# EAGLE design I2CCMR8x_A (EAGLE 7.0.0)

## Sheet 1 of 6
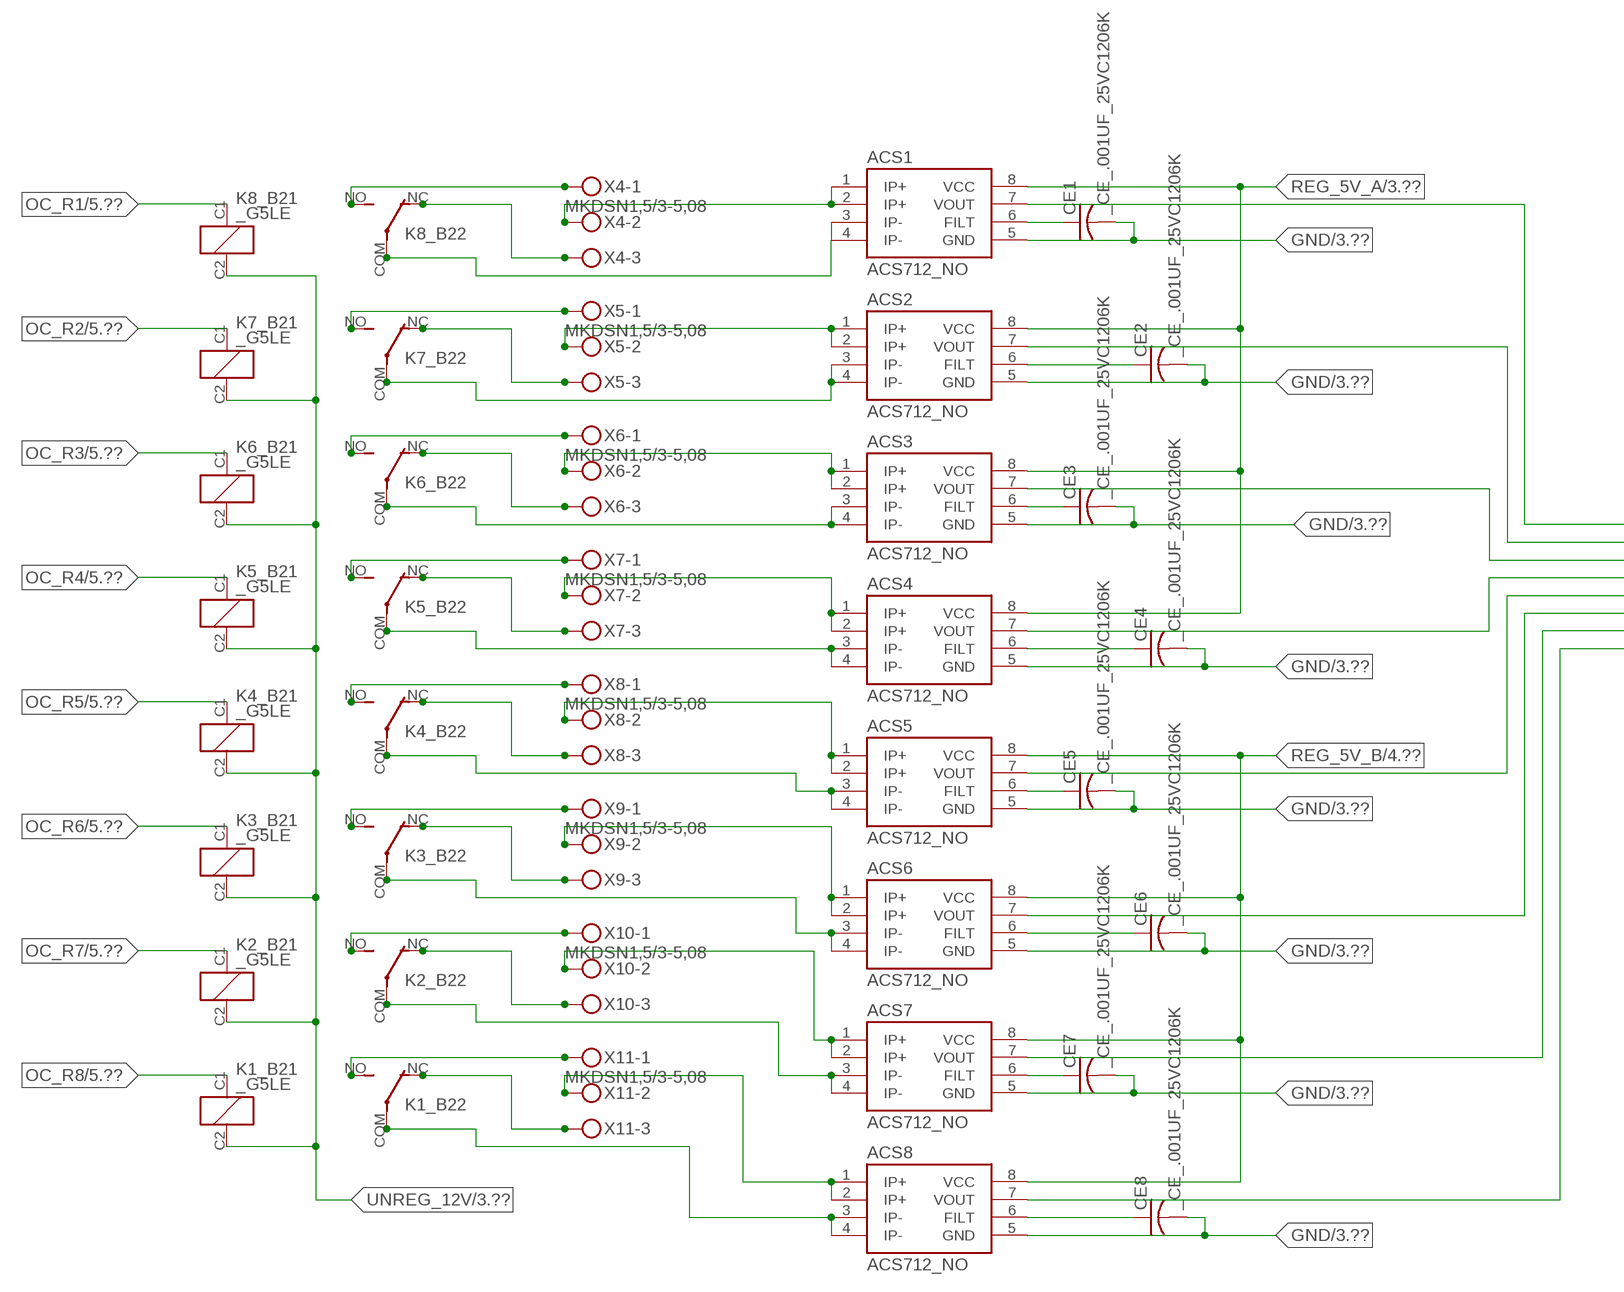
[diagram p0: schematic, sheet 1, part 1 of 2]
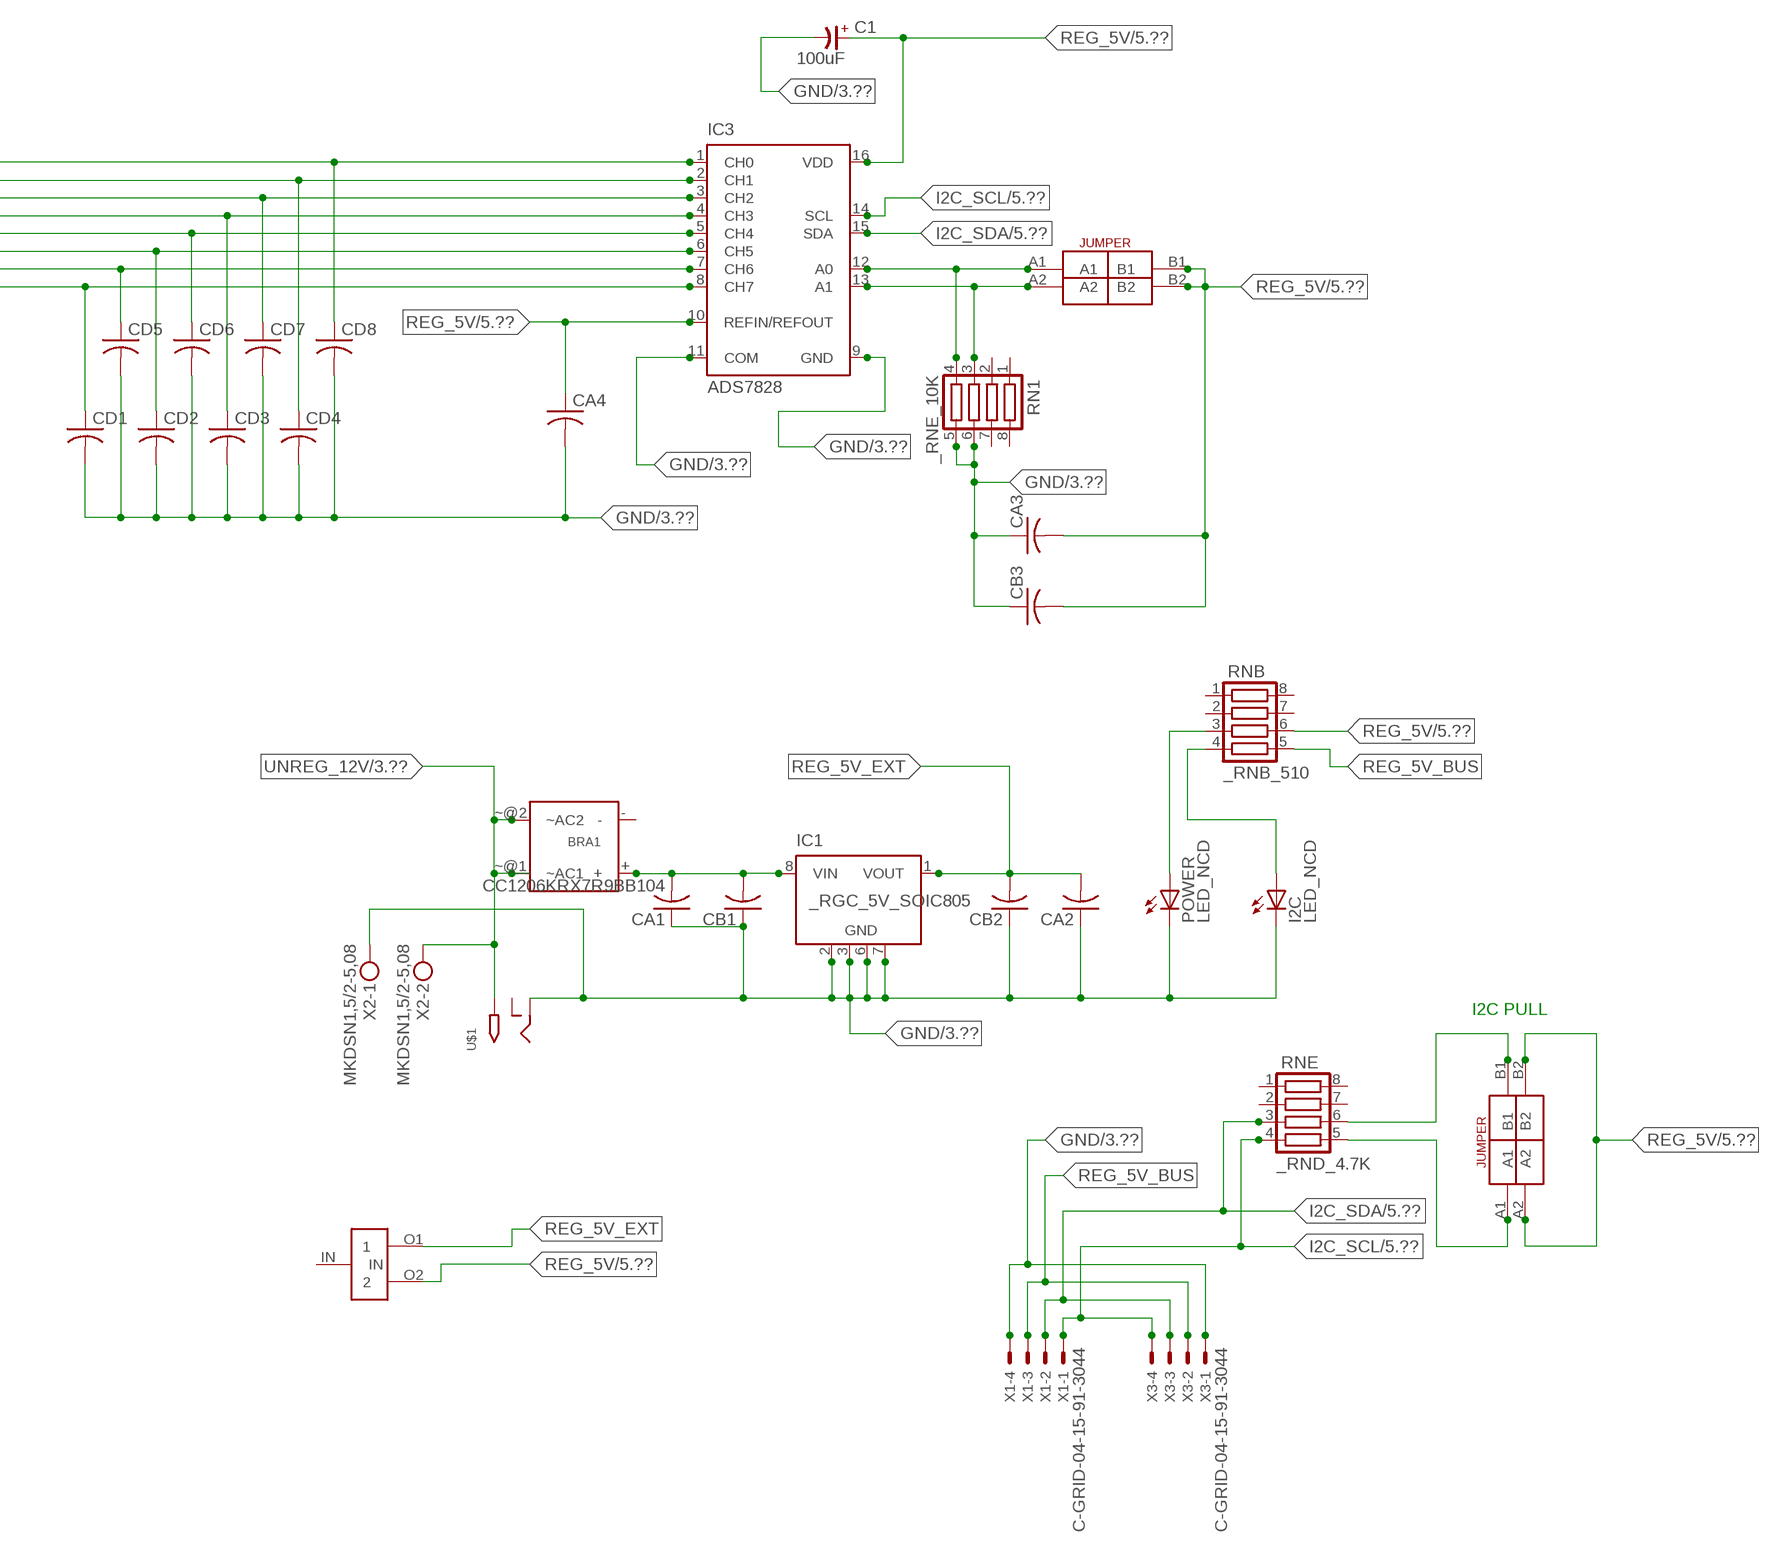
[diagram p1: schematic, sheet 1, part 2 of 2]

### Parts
ACS1  ACS712_NO  [_MA_DUAL_N-FET]
ACS2  ACS712_NO  [_MA_DUAL_N-FET]
ACS3  ACS712_NO  [_MA_DUAL_N-FET]
ACS4  ACS712_NO  [_MA_DUAL_N-FET]
ACS5  ACS712_NO  [_MA_DUAL_N-FET]
ACS6  ACS712_NO  [_MA_DUAL_N-FET]
ACS7  ACS712_NO  [_MA_DUAL_N-FET]
ACS8  ACS712_NO  [_MA_DUAL_N-FET]
BRA1  MB2S_  [MB2S]
C1  100uF  CP-E-025X060  [E-025X060]
CA1  CC1206KRX7R9BB104  [.1UF]
CA2  CC1206KRX7R9BB104C1206K  [CC1206KRX7R9BB104]
CA3  CC1206KRX7R9BB104C1206K  [CC1206KRX7R9BB104]
CA4  CC1206KRX7R9BB104C1206K  [CC1206KRX7R9BB104]
CB1  TMK316F106ZL-TC1206K  [TMK316F106ZL-T]
CB2  TMK316F106ZL-TC1206K  [TMK316F106ZL-T]
CB3  TMK316F106ZL-TC1206K  [TMK316F106ZL-T]
CD1  _CD_10NF_50VC1206K  [_CD_10NF_50V]
CD2  _CD_10NF_50VC1206K  [_CD_10NF_50V]
CD3  _CD_10NF_50VC1206K  [_CD_10NF_50V]
CD4  _CD_10NF_50VC1206K  [_CD_10NF_50V]
CD5  _CD_10NF_50VC1206K  [_CD_10NF_50V]
CD6  _CD_10NF_50VC1206K  [_CD_10NF_50V]
CD7  _CD_10NF_50VC1206K  [_CD_10NF_50V]
CD8  _CD_10NF_50VC1206K  [_CD_10NF_50V]
CE1  _CE_.001UF_25VC1206K  [CE]
CE2  _CE_.001UF_25VC1206K  [CE]
CE3  _CE_.001UF_25VC1206K  [CE]
CE4  _CE_.001UF_25VC1206K  [CE]
CE5  _CE_.001UF_25VC1206K  [CE]
CE6  _CE_.001UF_25VC1206K  [CE]
CE7  _CE_.001UF_25VC1206K  [CE]
CE8  _CE_.001UF_25VC1206K  [CE]
I2C  LED_NCD  [CHIPLED_0603]
IC1  _RGC_5V_SOIC805  [_RGC_5V_SOIC8]
IC3  ADS7828  [TSSOP16-PW]
K1_B2  _G5LE  [G5LE]
K2_B2  _G5LE  [G5LE]
K3_B2  _G5LE  [G5LE]
K4_B2  _G5LE  [G5LE]
K5_B2  _G5LE  [G5LE]
K6_B2  _G5LE  [G5LE]
K7_B2  _G5LE  [G5LE]
K8_B2  _G5LE  [G5LE]
POWER  LED_NCD  [CHIPLED_0603]
RN1  _RNE_10K  [RNE]
RNB  _RNB_510  [RNB]
RNE  _RND_4.7K  [RND]
U$1  2.1MMJACK  [PJ-102A]
U$2  LINK_2  [LINK_2]
U$3  JUMPER_2X2  [JUMPER_2X2]
U$4  JUMPER_2X2  [JUMPER_2X2]
X1  C-GRID-04-15-91-3044  [15-91-04]
X2  MKDSN1,5/2-5,08  [MKDSN1,5/2-5,08]
X3  C-GRID-04-15-91-3044  [15-91-04]
X4  MKDSN1,5/3-5,08  [MKDSN1,5/3-5,08]
X5  MKDSN1,5/3-5,08  [MKDSN1,5/3-5,08]
X6  MKDSN1,5/3-5,08  [MKDSN1,5/3-5,08]
X7  MKDSN1,5/3-5,08  [MKDSN1,5/3-5,08]
X8  MKDSN1,5/3-5,08  [MKDSN1,5/3-5,08]
X9  MKDSN1,5/3-5,08  [MKDSN1,5/3-5,08]
X10  MKDSN1,5/3-5,08  [MKDSN1,5/3-5,08]
X11  MKDSN1,5/3-5,08  [MKDSN1,5/3-5,08]

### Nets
GND: ACS1.5(GND) ACS2.5(GND) ACS3.5(GND) ACS4.5(GND) ACS5.5(GND) ACS6.5(GND) ACS7.5(GND) ACS8.5(GND) C1.- CA1.1 CA2.1 CA3.1 CA4.2 CB1.1 CB2.1 CB3.1 CD1.2 CD2.2 CD3.2 CD4.2 CD5.2 CD6.2 CD7.2 CD8.2 CE1.2 CE2.2 CE3.2 CE4.2 CE5.2 CE6.2 CE7.2 CE8.2 I2C.C IC1.2(GND) IC1.3(GND) IC1.6(GND) IC1.7(GND) IC3.9(GND) IC3.11(COM) POWER.C RN1.5 RN1.6 U$1.RING X1.4 X2.1 X3.1 ; also sheet 3,4,5
I2C_SCL: IC3.14(SCL) RNE.4 X1.1 X3.4 ; also sheet 5
I2C_SDA: IC3.15(SDA) RNE.3 X1.2 X3.3 ; also sheet 5
N$1: BRA1.+ CA1.2 CB1.2 IC1.8(VIN)
N$2: POWER.A RNB.3
N$3: I2C.A RNB.4
N$4: RNE.5 U$3.A1
N$5: RNE.6 U$3.B1
N$6: ACS5.7(VOUT) CD6.1 IC3.5(CH4)
N$7: ACS1.1(IP+) ACS1.2(IP+) X4.2
N$9: ACS1.7(VOUT) CD8.1 IC3.1(CH0)
N$10: ACS2.7(VOUT) CD4.1 IC3.2(CH1)
N$11: ACS3.7(VOUT) CD7.1 IC3.3(CH2)
N$12: ACS4.7(VOUT) CD3.1 IC3.4(CH3)
N$13: ACS2.1(IP+) ACS2.2(IP+) X5.2
N$14: ACS6.7(VOUT) CD2.1 IC3.6(CH5)
N$15: ACS7.7(VOUT) CD5.1 IC3.7(CH6)
N$17: IC3.12(A0) RN1.4 U$4.A1
N$18: IC3.13(A1) RN1.3 U$4.A2
N$21: ACS4.1(IP+) ACS4.2(IP+) X7.2
N$22: ACS4.3(IP-) ACS4.4(IP-) K5_B2.COM(2:COM)
N$23: ACS5.1(IP+) ACS5.2(IP+) X8.2
N$24: ACS7.1(IP+) ACS7.2(IP+) X10.2
N$25: ACS6.1(IP+) ACS6.2(IP+) X9.2
N$29: ACS8.1(IP+) ACS8.2(IP+) X11.2
N$33: ACS1.6(FILT) CE1.1
N$34: ACS2.6(FILT) CE2.1
N$35: ACS3.6(FILT) CE3.1
N$36: ACS4.6(FILT) CE4.1
N$37: ACS8.7(VOUT) CD1.1 IC3.8(CH7)
N$38: ACS5.6(FILT) CE5.1
N$39: ACS6.6(FILT) CE6.1
N$40: ACS7.6(FILT) CE7.1
N$41: ACS8.6(FILT) CE8.1
N$42: ACS1.3(IP-) ACS1.4(IP-) K8_B2.COM(2:COM)
N$43: K8_B2.NC(2:NC) X4.3
N$44: K8_B2.NO(2:NO) X4.1
N$45: K7_B2.NO(2:NO) X5.1
N$46: K6_B2.NO(2:NO) X6.1
N$137: K7_B2.NC(2:NC) X5.3
N$138: ACS2.3(IP-) ACS2.4(IP-) K7_B2.COM(2:COM)
N$139: K6_B2.NC(2:NC) X6.3
N$140: ACS3.3(IP-) ACS3.4(IP-) K6_B2.COM(2:COM)
N$141: K5_B2.NC(2:NC) X7.3
N$143: K5_B2.NO(2:NO) X7.1
N$144: K4_B2.NO(2:NO) X8.1
N$145: K4_B2.NC(2:NC) X8.3
N$146: ACS5.3(IP-) ACS5.4(IP-) K4_B2.COM(2:COM)
N$147: K3_B2.NO(2:NO) X9.1
N$148: K3_B2.NC(2:NC) X9.3
N$149: ACS6.3(IP-) ACS6.4(IP-) K3_B2.COM(2:COM)
N$150: K2_B2.NO(2:NO) X10.1
N$151: K2_B2.NC(2:NC) X10.3
N$152: ACS7.3(IP-) ACS7.4(IP-) K2_B2.COM(2:COM)
N$153: K1_B2.NO(2:NO) X11.1
N$154: K1_B2.NC(2:NC) X11.3
N$155: ACS8.3(IP-) ACS8.4(IP-) K1_B2.COM(2:COM)
N$166: ACS3.1(IP+) ACS3.2(IP+) X6.2
OC_R1: K8_B2.C1(1:C1) ; also sheet 5
OC_R2: K7_B2.C1(1:C1) ; also sheet 5
OC_R3: K6_B2.C1(1:C1) ; also sheet 5
OC_R4: K5_B2.C1(1:C1) ; also sheet 5
OC_R5: K4_B2.C1(1:C1) ; also sheet 5
OC_R6: K3_B2.C1(1:C1) ; also sheet 5
OC_R7: K2_B2.C1(1:C1) ; also sheet 5
OC_R8: K1_B2.C1(1:C1) ; also sheet 5
REG_5V: C1.+ CA3.2 CA4.1 CB3.2 IC3.10(REFIN/REFOUT) IC3.16(VDD) RNB.6 U$2.O2 U$3.A2 U$3.B2 U$4.B1 U$4.B2 ; also sheet 5
REG_5V_A: ACS1.8(VCC) ACS2.8(VCC) ACS3.8(VCC) ACS4.8(VCC) ; also sheet 3
REG_5V_B: ACS5.8(VCC) ACS6.8(VCC) ACS7.8(VCC) ACS8.8(VCC) ; also sheet 4
REG_5V_BUS: RNB.5 X1.3 X3.2
REG_5V_EXT: CA2.2 CB2.2 IC1.1(VOUT) U$2.O1
UNREG_12V: BRA1.~@1(~AC1) BRA1.~@2(~AC2) K1_B2.C2(1:C2) K2_B2.C2(1:C2) K3_B2.C2(1:C2) K4_B2.C2(1:C2) K5_B2.C2(1:C2) K6_B2.C2(1:C2) K7_B2.C2(1:C2) K8_B2.C2(1:C2) U$1.TIP X2.2 ; also sheet 3,4,5
Unconnected: BRA1.- IC1.4(NC) IC1.5(NC) RN1.1 RN1.2 RN1.7 RN1.8 RNB.1 RNB.2 RNB.7 RNB.8 RNE.1 RNE.2 RNE.7 RNE.8 U$1.RING_SW U$2.IN

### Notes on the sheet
- I2C PULL

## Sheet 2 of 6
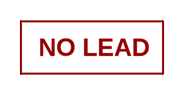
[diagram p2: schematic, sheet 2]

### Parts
U$16  NOPB_LOGO_SYM  [NOPB_LOGO_SYM]

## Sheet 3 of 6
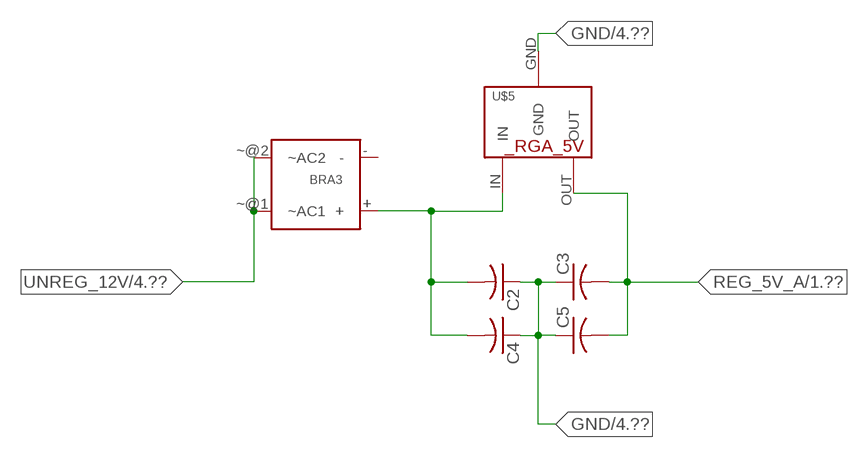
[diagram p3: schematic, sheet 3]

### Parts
BRA3  MB2S_  [MB2S]
C2  _CA_.10UF_50VC1206K  [_CA_.1UF_50V]
C3  _CA_.10UF_50VC1206K  [_CA_.1UF_50V]
C4  _CB_10UF_25VC1206K  [_CB_10UF_25V]
C5  _CB_10UF_25VC1206K  [_CB_10UF_25V]
U$5  _RGA_5V  [_RGA_5V]

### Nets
GND: C2.1 C3.1 C4.1 C5.1 U$5.GND ; also sheet 1,4,5
N$31: BRA3.+ C2.2 C4.2 U$5.IN
REG_5V_A: C3.2 C5.2 U$5.OUT ; also sheet 1
UNREG_12V: BRA3.~@1(~AC1) BRA3.~@2(~AC2) ; also sheet 1,4,5
Unconnected: BRA3.-

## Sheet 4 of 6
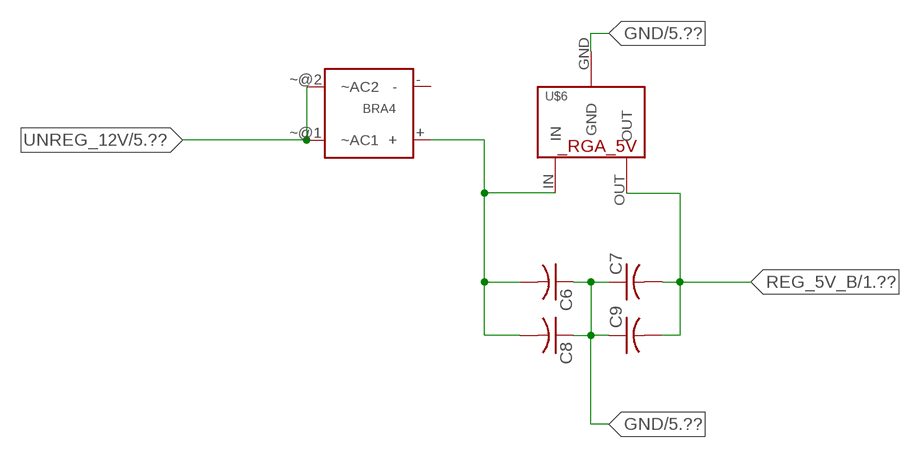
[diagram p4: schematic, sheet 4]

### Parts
BRA4  MB2S_  [MB2S]
C6  _CA_.10UF_50VC1206K  [_CA_.1UF_50V]
C7  _CA_.10UF_50VC1206K  [_CA_.1UF_50V]
C8  _CB_10UF_25VC1206K  [_CB_10UF_25V]
C9  _CB_10UF_25VC1206K  [_CB_10UF_25V]
U$6  _RGA_5V  [_RGA_5V]

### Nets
GND: C6.1 C7.1 C8.1 C9.1 U$6.GND ; also sheet 1,3,5
N$32: BRA4.+ C6.2 C8.2 U$6.IN
REG_5V_B: C7.2 C9.2 U$6.OUT ; also sheet 1
UNREG_12V: BRA4.~@1(~AC1) BRA4.~@2(~AC2) ; also sheet 1,3,5
Unconnected: BRA4.-

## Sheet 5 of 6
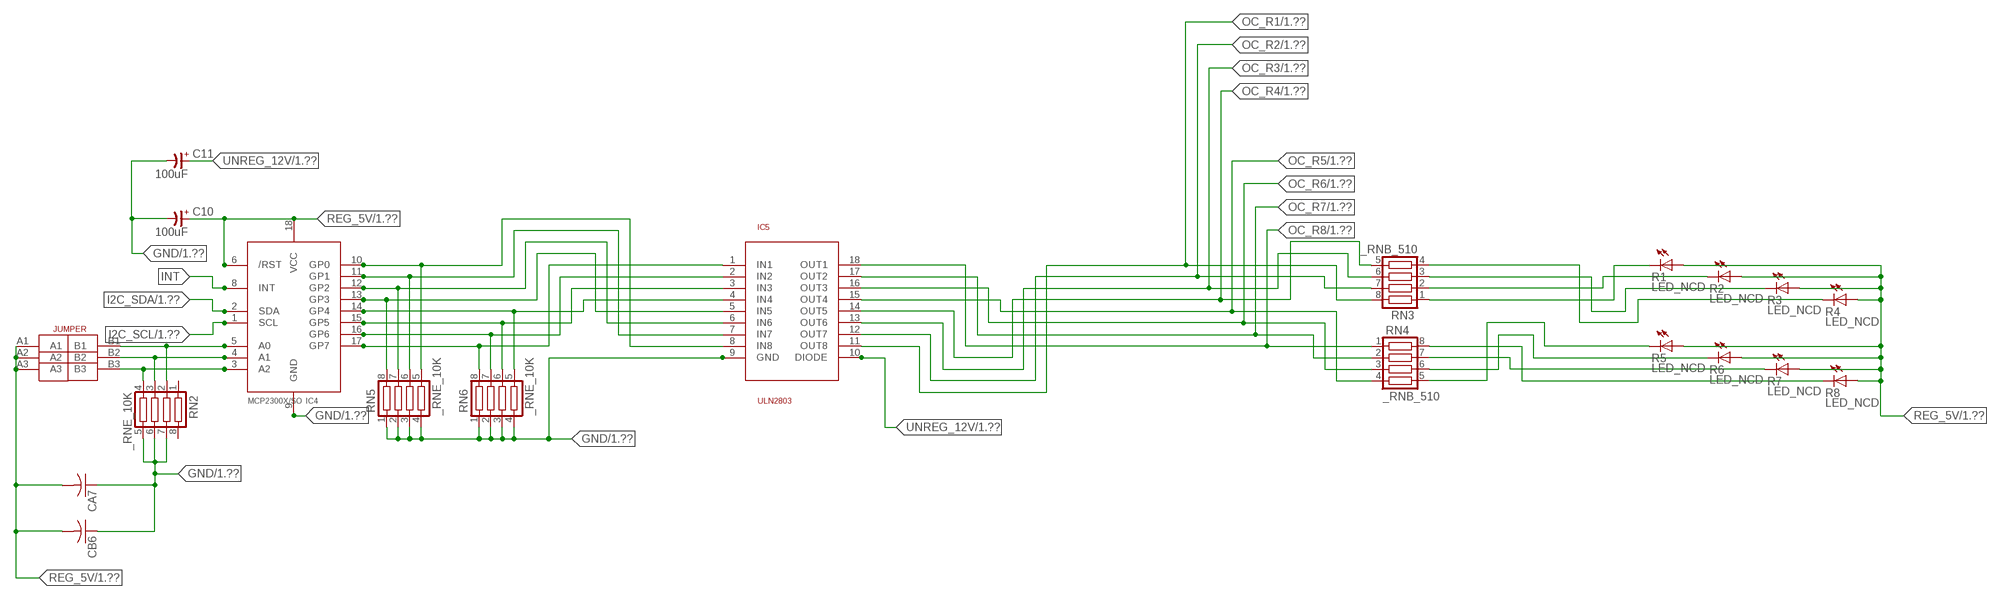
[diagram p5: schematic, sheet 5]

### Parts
C10  100uF  CP-E-025X060  [E-025X060]
C11  100uF  CP-E-025X060  [E-025X060]
CA7  CC1206KRX7R9BB104C1206K  [CC1206KRX7R9BB104]
CB6  TMK316F106ZL-TC1206K  [TMK316F106ZL-T]
IC4  MCP2300X/SO  [SO18W]
IC5  ULN2803  [SO18L]
R1  LED_NCD  [CHIPLED_0603]
R2  LED_NCD  [CHIPLED_0603]
R3  LED_NCD  [CHIPLED_0603]
R4  LED_NCD  [CHIPLED_0603]
R5  LED_NCD  [CHIPLED_0603]
R6  LED_NCD  [CHIPLED_0603]
R7  LED_NCD  [CHIPLED_0603]
R8  LED_NCD  [CHIPLED_0603]
RN2  _RNE_10K  [RNE]
RN3  _RNB_510  [RNB]
RN4  _RNB_510  [RNB]
RN5  _RNE_10K  [RNE]
RN6  _RNE_10K  [RNE]
U$18  JUMPER_3X2  [JUMPER_3X2]

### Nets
GND: C10.- C11.- CA7.1 CB6.1 IC4.9(GND) IC5.9(GND) RN2.5 RN2.6 RN2.7 RN5.1 RN5.2 RN5.3 RN5.4 RN6.1 RN6.2 RN6.3 RN6.4 ; also sheet 1,3,4
GP4: IC4.14(GP4) IC5.4(IN4) RN6.5
GP6: IC4.16(GP6) IC5.2(IN2) RN6.7
I2C_SCL: IC4.1(SCL) ; also sheet 1
I2C_SDA: IC4.2(SDA) ; also sheet 1
INT: IC4.8(INT)
N$47: IC4.5(A0) RN2.2 U$18.B1
N$48: IC4.4(A1) RN2.3 U$18.B2
N$49: IC4.3(A2) RN2.4 U$18.B3
N$50: IC4.12(GP2) IC5.6(IN6) RN5.7
N$51: IC4.11(GP1) IC5.7(IN7) RN5.6
N$52: IC4.10(GP0) IC5.8(IN8) RN5.5
N$53: R1.C RN3.1
N$54: R2.C RN3.2
N$55: R3.C RN3.3
N$56: R4.C RN3.4
N$57: R8.C RN4.8
N$81: R7.C RN4.7
N$82: R6.C RN4.6
N$83: R5.C RN4.5
N$89: IC4.13(GP3) IC5.5(IN5) RN5.8
N$93: IC4.15(GP5) IC5.3(IN3) RN6.6
N$94: IC4.17(GP7) IC5.1(IN1) RN6.8
OC_R1: IC5.11(OUT8) RN3.8 ; also sheet 1
OC_R2: IC5.12(OUT7) RN3.7 ; also sheet 1
OC_R3: IC5.13(OUT6) RN3.6 ; also sheet 1
OC_R4: IC5.14(OUT5) RN3.5 ; also sheet 1
OC_R5: IC5.15(OUT4) RN4.4 ; also sheet 1
OC_R6: IC5.16(OUT3) RN4.3 ; also sheet 1
OC_R7: IC5.17(OUT2) RN4.2 ; also sheet 1
OC_R8: IC5.18(OUT1) RN4.1 ; also sheet 1
REG_5V: C10.+ CA7.2 CB6.2 IC4.6(/RST) IC4.18(VCC) R1.A R2.A R3.A R4.A R5.A R6.A R7.A R8.A U$18.A1 U$18.A2 U$18.A3 ; also sheet 1
UNREG_12V: C11.+ IC5.10(DIODE) ; also sheet 1,3,4
Unconnected: RN2.1 RN2.8

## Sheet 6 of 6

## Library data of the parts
ACS1-ACS8 = NCD_ULTIMATE_LIBRARY:ACS712_NO: Semiconductor Sensor Current Hall-effect-based isolated linear current sensor Digikey 620-1190-2-ND/ACS712ELCTR-20A-T
BRA1 BRA3 BRA4 = NCD_ULTIMATE_LIBRARY:MB2S: Bridge Rectifier BRA MB2S 200V 500ma Digikey MB2S-TPMSTR-ND/MB2S-TP
C1 C10 C11 = NCD_ULTIMATE_LIBRARY:CP-: Capacitors All Kinds POLARIZED CAP
C2 C3 C6 C7 = NCD_ULTIMATE_LIBRARY:_CA_.10UF_50V: Capacitor .1uF SMT
C4 C5 C8 C9 = NCD_ULTIMATE_LIBRARY:_CB_10UF_25V: Capacitor 10uF SMT
CA1-CA4 CA7 = NCD_ULTIMATE_LIBRARY:CC1206KRX7R9BB104: Capacitor CA .1uF 50V SMT C1206K CC1206KRX7R9BB104
CB1-CB3 CB6 = NCD_ULTIMATE_LIBRARY:TMK316F106ZL-T: Capacitor CB 10uF SMT 1206 TMK316F106ZL-T
CD1-CD8 = NCD_ULTIMATE_LIBRARY:_CD_10NF_50V: Capacitor 10nF SMT
CE1-CE8 = NCD_ULTIMATE_LIBRARY:_CE_.001UF_25V: Capacitor .001uF SMT
I2C POWER = NCD_ULTIMATE_bhaskar:LED_NCD
IC1 = NCD_ULTIMATE_LIBRARY:_RGC_5V_SOIC8: Regulator Linear 5V Chip Positive VOLTAGE REGULATOR Digikey 497-7267-2-ND/L78L05CD13TR
IC3 = NCD_ULTIMATE_LIBRARY:ADS7828: Semiconductor ADC I2C 12-Bit, 8-Channel Sampling ANALOG-TO-DIGITAL CONVERTER Digikey 296-12402-2-ND Source: www.ti.com .. ADS7828.pdf / ADS7828E/250; MF: TEXAS INSTRUMENTS; MPN: ADS7828E/250; OC_FARNELL: 1470338; OC_NEWARK: 74C7158
IC4 = NCD_ULTIMATE_LIBRARY:MCP2300X: Semiconductor Port Expander I/O 8-Bit I2C MCP23008 Inexpensive i2c i/o expander - 8 general purpose i/o pins with optional pullups
IC5 = NCD_ULTIMATE_LIBRARY:ULN2803: Semiconductor 8 O.C. N-Channel Transistor Driver Digikey ULN2803AFWGCELTR-ND/ULN2803AFWG,C,EL
K1_B2 K2_B2 K3_B2 K4_B2 K5_B2 K6_B2 K7_B2 K8_B2 = NCD_ULTIMATE_LIBRARY:_G5LE: Relay 5A/10A SPDT; OC_FARNELL: unknown; OC_NEWARK: unknown
R1-R8 = NCD_ULTIMATE_LIBRARY:LED_NCD: LED Digikey 754-1132-2-ND/APT2012SRCPRV
RN1 RN2 RN5 RN6 = NCD_ULTIMATE_LIBRARY:_RNE_10K: Resistor Array RNE SMT 10K x 4 Single Resistor Source: http://www.ctscorp.com/components/Datasheets/CTSChipArrayDs.pdf Digikey 742C083103JPTR-ND/742C083103JP; OC_FARNELL: unknown; OC_NEWARK: unknown
RN3 RN4 RNB = NCD_ULTIMATE_LIBRARY:_RNB_510: Resistor Array RNB SMT 510 x 4 Single Resistor Source: http://www.ctscorp.com/components/Datasheets/CTSChipArrayDs.pdf Digikey 742C083511JPTR-ND/ 742C083511JP; OC_FARNELL: unknown; OC_NEWARK: unknown
RNE = NCD_ULTIMATE_LIBRARY:_RND_4.7K: Resistor Array RND SMT 4.7K x 4 Single Resistor Source: http://www.ctscorp.com/components/Datasheets/CTSChipArrayDs.pdf Digikey 742C083472JPTR-ND/742C083472JP; OC_FARNELL: unknown; OC_NEWARK: unknown
U$1 = NCD_ULTIMATE_CONNECTORS:2.1MMJACK: 2.1mm x 5.5mm DC jack with internal switch. Digikey part #PJ-102A, 4UCON part #05537 By microbuilder.eu
U$2 = NCD_ULTIMATE_LIBRARY:LINK_2: PAD_top
U$3 U$4 = NCD_ULTIMATE_CONNECTORS:JUMPER_2X2
U$5 U$6 = NCD_ULTIMATE_LIBRARY:_RGA_5V: Regulator Linear 5V Digikey 497-7255-2-ND/ L7805CDT-TR
U$16 = PatternAgents-Logos:NOPB_LOGO_SYM: NOPB_LOGO_SYM
U$18 = NCD_ULTIMATE_CONNECTORS:JUMPER_3X2
X1 X3 = NCD_ULTIMATE_CONNECTORS:C-GRID-04: CONNECTOR 4-Pos I2C wire to board 2.54 mm (0.100") pitch header Digikey WM1342-ND/0015912045; OC_FARNELL: unknown; OC_NEWARK: unknown
X2 = NCD_ULTIMATE_CONNECTORS:MKDSN1,5/2-5,08: MKDSN 1,5/ 2-5,08 Printklemme
X4-X11 = NCD_ULTIMATE_CONNECTORS:MKDSN1,5/3-5,08: MKDSN 1,5/ 3-5,08 Printklemme Nennstrom: 13,5 A Nennspannung: 250 V Rastermaß: 5,08 mm Polzahl: 3 Anschlussart: Schraubanschluss Montage: Löten Anschlussrichtung Leiter/Platine: 0 ° Artikelnummer: 1729131 Source: http://eshop.phoenixcontact.com .. 1729131.pdf

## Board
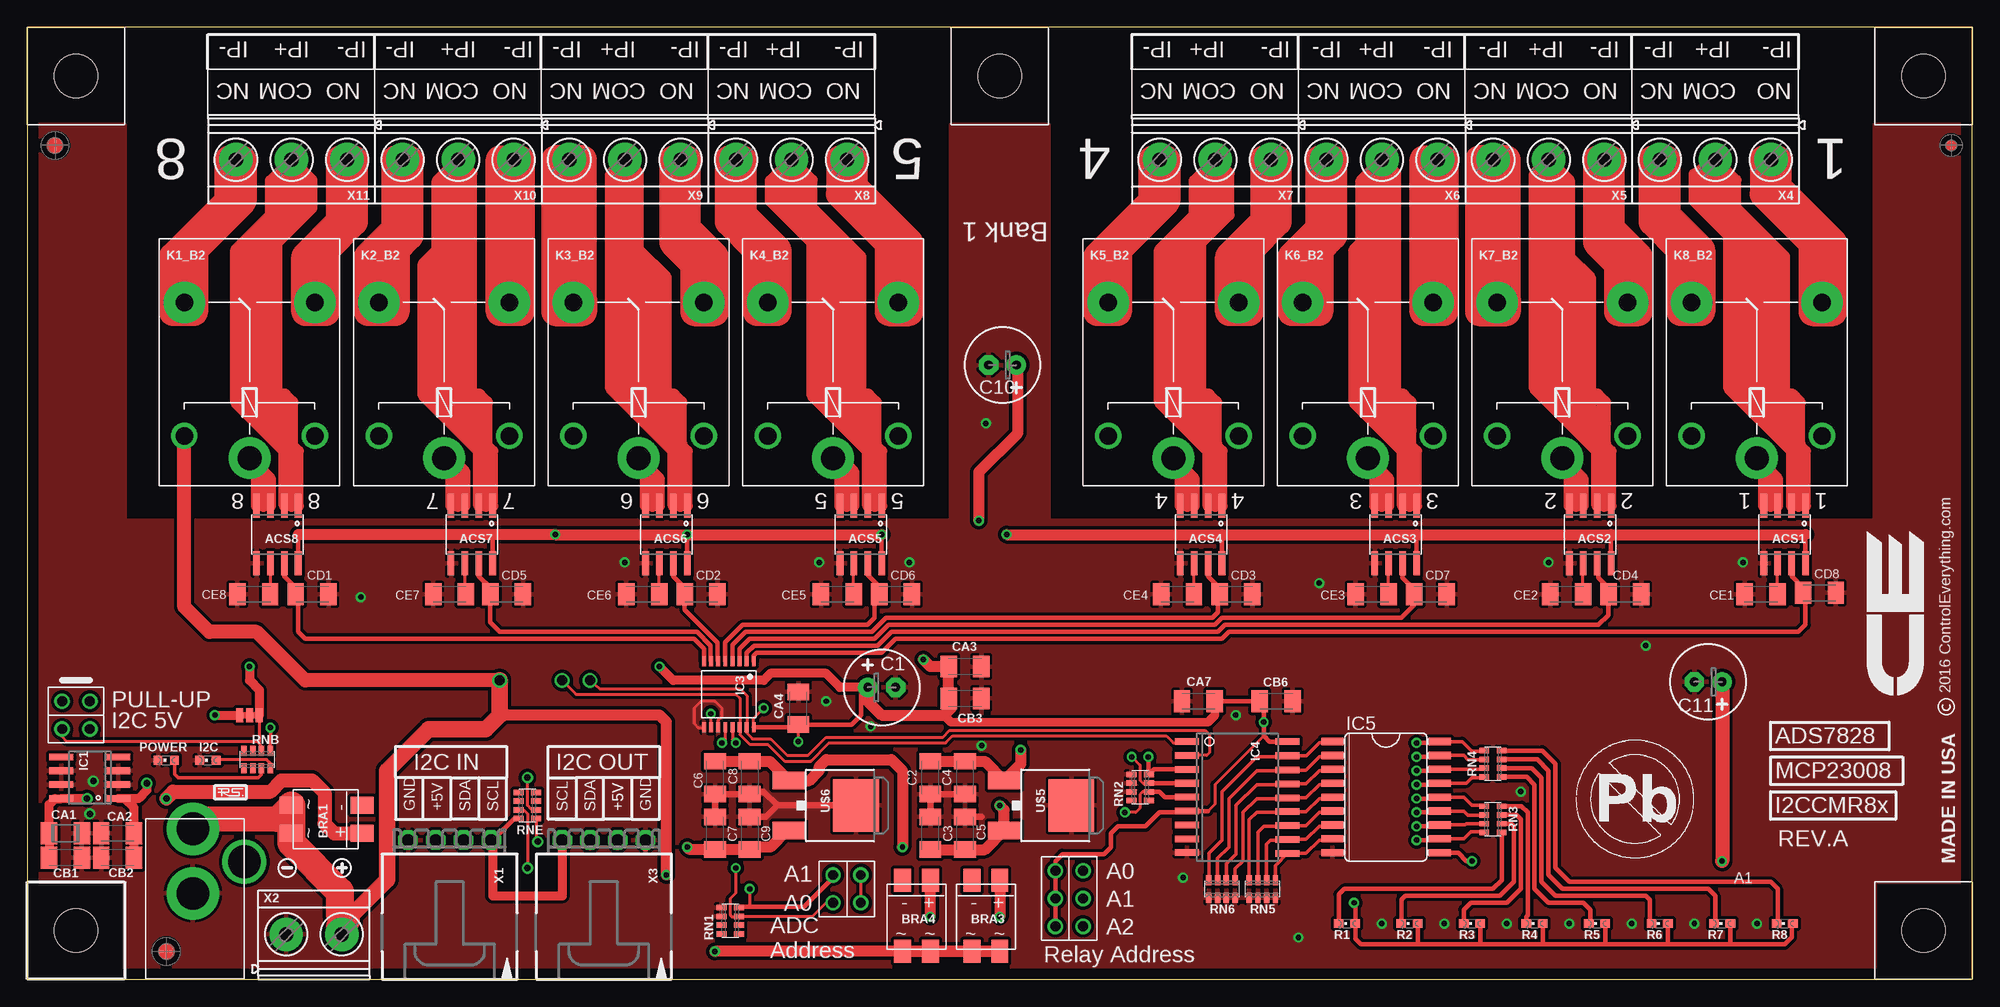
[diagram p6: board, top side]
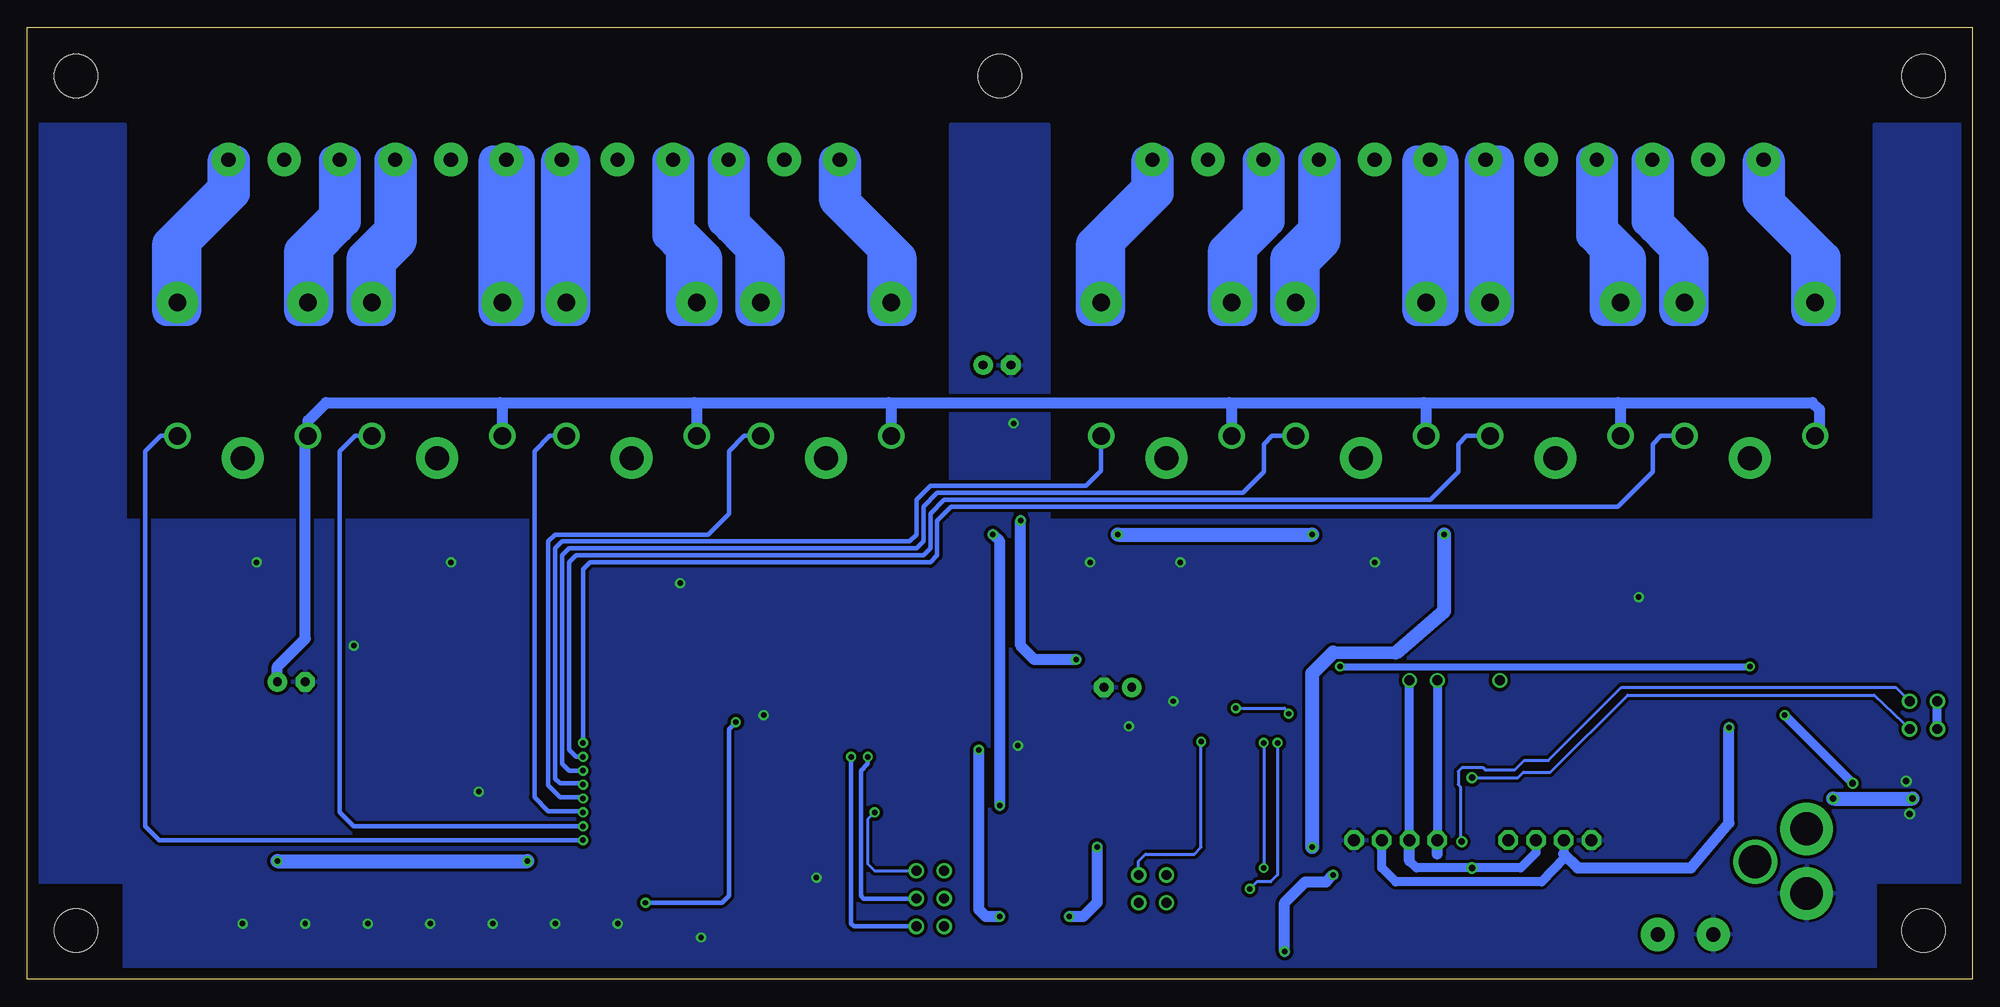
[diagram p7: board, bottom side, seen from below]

Size 177.8 x 87 mm. Coordinates in mm from the lower left corner, seen from the top.
Outline: 0,86.67 0,85.72
Outline: 0,85.72 0,0 177.8,0 177.8,87 0,87 0,85.72
Copper layers (1*16): Top 0.035mm / dielectric 1.5mm / Bottom 0.035mm
Design rules "default": minimum track width 10mil, minimum drill 24mil, track to track 8mil, track to pad 8mil, pad to pad 8mil, via to via 8mil, smd to smd 8mil, copper to edge 40mil, drill to drill 8mil, minimum pad ring 10mil, minimum via ring 8mil, stop-mask expansion 4mil, vias tented up to drill 0mil, thermal gap 10mil
Holes 3.96 mm at 4.45,4.45

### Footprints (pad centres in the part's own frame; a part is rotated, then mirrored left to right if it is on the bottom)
_MA_DUAL_N-FET = smd 0.61 x 2.21: 1 -1.905,-2.616; 2 -0.635,-2.616; 3 0.635,-2.616; 4 1.905,-2.616; 5 1.905,2.616; 6 0.635,2.616; 7 -0.635,2.616; 8 -1.905,2.616
MB2S = smd 1.55 x 2.1: + 0,-6.5; - 2.54,-6.5; ~@1 0,0; ~@2 2.54,0
E-025X060 = drill 0.813 pad 1.778: + -1.27,0 | drill 0.813 pad 1.778 octagon: - 1.27,0
_CA_.1UF_50V = smd 1.5 x 2: 1 -1.5,0; 2 1.5,0
_CB_10UF_25V = smd 1.5 x 2: 1 -1.5,0; 2 1.5,0
.1UF = smd 1.5 x 2: 1 -1.5,0; 2 1.5,0
CC1206KRX7R9BB104 = smd 1.5 x 2: 1 -1.5,0; 2 1.5,0
TMK316F106ZL-T = smd 1.5 x 2: 1 -1.5,0; 2 1.5,0
_CD_10NF_50V = smd 1.5 x 2: 1 -1.5,0; 2 1.5,0
CE = smd 1.5 x 2: 1 -1.5,0; 2 1.5,0
CHIPLED_0603 = smd 0.8 x 0.8: A 0,-0.75; C 0,0.75
_RGC_5V_SOIC8 = smd 0.6 x 2.2: 1 -1.905,-2.6; 2 -0.635,-2.6; 3 0.635,-2.6; 4 1.905,-2.6; 5 1.905,2.6; 6 0.635,2.6; 7 -0.635,2.6; 8 -1.905,2.6
TSSOP16-PW = smd 0.35 x 0.9: 1 -2.275,-3.025; 2 -1.625,-3.025; 3 -0.975,-3.025; 4 -0.325,-3.025; 5 0.325,-3.025; 6 0.975,-3.025; 7 1.625,-3.025; 8 2.275,-3.025; 9 2.275,3.025; 10 1.625,3.025; 11 0.975,3.025; 12 0.325,3.025; 13 -0.325,3.025; 14 -0.975,3.025; 15 -1.625,3.025; 16 -2.275,3.025
SO18W = smd 0.6 x 2.2: 1 -4.445,-4.6; 2 -3.175,-4.6; 3 -1.905,-4.6; 4 -0.635,-4.6; 5 0.635,-4.6; 6 1.905,-4.6; 7 3.175,-4.6; 8 4.445,-4.6; 9 5.715,-4.6; 10 5.775,4.6; 11 4.505,4.6; 12 3.235,4.6; 13 1.965,4.6; 14 0.695,4.6; 15 -0.575,4.6; 16 -1.845,4.6; 17 -3.145,4.6; 18 -4.445,4.6
SO18L = smd 0.66 x 2.032: 1 -5.08,-4.902; 2 -3.81,-4.902; 3 -2.54,-4.902; 4 -1.27,-4.902; 5 0,-4.902; 6 1.27,-4.902; 7 2.54,-4.902; 8 3.81,-4.902; 9 5.08,-4.902; 10 5.08,4.902; 11 3.81,4.902; 12 2.54,4.902; 13 1.27,4.902; 14 0,4.902; 15 -1.27,4.902; 16 -2.54,4.902; 17 -3.81,4.902; 18 -5.08,4.902
G5LE = drill 1.6: C1 -7.493,-5.969; C2 -7.493,5.969 | drill 2.2 pad 3.81: COM -9.525,0 | drill 1.6 pad 3.81: NC 4.699,5.969; NO 4.699,-5.969
CHIPLED_0603' = smd 0.8 x 0.876: A 0,-0.75; C 0,0.75
RNE = smd 0.5 x 0.9: 1 -1.2,-0.8; 2 -0.4,-0.8; 3 0.4,-0.8; 4 1.2,-0.8; 5 1.2,0.8; 6 0.4,0.8; 7 -0.4,0.8; 8 -1.2,0.8
RNB = smd 0.5 x 0.9: 1 -1.2,-0.8; 2 -0.4,-0.8; 3 0.4,-0.8; 4 1.2,-0.8; 5 1.2,0.8; 6 0.4,0.8; 7 -0.4,0.8; 8 -1.2,0.8
RND = smd 0.5 x 0.9: 1 -1.2,-0.8; 2 -0.4,-0.8; 3 0.4,-0.8; 4 1.2,-0.8; 5 1.2,0.8; 6 0.4,0.8; 7 -0.4,0.8; 8 -1.2,0.8
PJ-102A = drill 3 pad 4.8: RING 0.1,-3.39; TIP 0.1,-9.29 | drill 3 pad 3.251: RING_SW -4.6,-6.29
LINK_2 = smd 1.27 x 0.635: IN 0,0; O1 0,0.889; O2 0,-0.889
JUMPER_2X2 = drill 0.9: A1 0,2.54; A2 0,0; B1 2.54,2.54; B2 2.54,0
_RGA_5V = smd 4.826 x 4.191: GND 0,2.096 | smd 1.6 x 3: IN -2.28,-4.04; OUT 2.28,-4.04
PCB_MOUNTING_HOLE = hole 3.962: 4.445,4.445
JUMPER_3X2 = drill 0.9: A1 0,5.08; A2 0,2.54; A3 0,0; B1 2.54,5.08; B2 2.54,2.54; B3 2.54,0
15-91-04 = drill 1.1 pad 1.778 octagon: 1 -3.81,-7.62; 2 -1.27,-7.62; 3 1.27,-7.62; 4 3.81,-7.62
MKDSN1,5/2-5,08 = drill 1.3 pad 3.048: 1 -2.561,0.025; 2 2.519,0.025
MKDSN1,5/3-5,08 = drill 1.3 pad 3.048: 1 -7.641,0.025; 2 -2.561,0.025; 3 2.519,0.025

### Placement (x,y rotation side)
ACS1  160.66,40.64 180 top
ACS2  142.88,40.64 180 top
ACS3  125.09,40.64 180 top
ACS4  107.31,40.64 180 top
ACS5  76.2,40.64 180 top
ACS6  58.42,40.64 180 top
ACS7  40.64,40.64 180 top
ACS8  22.86,40.64 180 top
BRA1  24.13,13.34 90 top
BRA3  88.9,2.54 180 top
BRA4  82.55,2.54 180 top
C1  78.11,26.67 0 top
C2  82.55,18.41 90 top
C3  82.55,13.34 270 top
C4  85.72,18.41 90 top
C5  85.72,13.34 270 top
C6  62.87,18.41 90 top
C7  62.87,13.34 270 top
C8  66.04,18.41 90 top
C9  66.04,13.34 270 top
C10  89.15,56.13 180 top
C11  153.67,27.18 180 top
CA1  3.49,13.34 180 top
CA2  8.26,13.34 0 top
CA3  85.72,28.57 180 top
CA4  70.48,24.77 90 top
CA7  107.06,25.4 0 top
CB1  3.49,11.11 180 top
CB2  8.26,11.11 0 top
CB3  85.72,25.65 180 top
CB6  114.17,25.4 180 top
CD1  26.04,35.18 0 top
CD2  61.59,35.18 0 top
CD3  110.49,35.18 0 top
CD4  146.05,35.18 0 top
CD5  43.81,35.18 0 top
CD6  79.38,35.18 0 top
CD7  128.27,35.18 0 top
CD8  163.83,35.31 0 top
CE1  158.5,35.18 180 top
CE2  140.72,35.18 180 top
CE3  122.94,35.18 180 top
CE4  105.16,35.18 180 top
CE5  74.04,35.18 180 top
CE6  56.26,35.18 180 top
CE7  38.61,35.18 180 top
CE8  20.7,35.18 180 top
I2C  16.51,20 90 top
IC1  5.71,18.41 90 top
IC3  64.14,26.04 180 top
IC4  110.62,17.27 270 top
IC5  124.21,16.64 270 top
K1_B2  20.32,57.15 90 top
K2_B2  38.1,57.15 90 top
K3_B2  55.88,57.15 90 top
K4_B2  73.66,57.15 90 top
K5_B2  104.78,57.15 90 top
K6_B2  122.56,57.15 90 top
K7_B2  140.34,57.15 90 top
K8_B2  158.12,57.15 90 top
POWER  12.7,20 90 top
R1  LED_NCD  [CHIPLED_0603']  120.65,5.08 90 top
R2  LED_NCD  [CHIPLED_0603']  126.36,5.08 90 top
R3  LED_NCD  [CHIPLED_0603']  132.08,5.08 90 top
R4  LED_NCD  [CHIPLED_0603']  137.79,5.08 90 top
R5  LED_NCD  [CHIPLED_0603']  143.51,5.08 90 top
R6  LED_NCD  [CHIPLED_0603']  149.22,5.08 90 top
R7  LED_NCD  [CHIPLED_0603']  154.94,5.08 90 top
R8  LED_NCD  [CHIPLED_0603']  160.66,5.08 90 top
RN1  64.26,5.33 90 top
RN2  101.73,17.53 90 top
RN3  133.99,14.61 90 top
RN4  133.99,19.68 270 top
RN5  112.9,8.26 0 top
RN6  109.22,8.26 0 top
RNB  21.02,20.07 0 top
RNE  45.72,15.88 270 top
U$1  15.24,4.45 180 top
U$2  20.32,24.13 90 top
U$3  3.17,25.4 270 top
U$4  73.66,6.99 0 top
U$5  93.34,15.88 270 top
U$6  73.66,15.88 270 top
U$10  [VISION_REF15]  12.7,2.54 0 top
U$15  PCB_MOUNTING_HOLE  [PCB_MOUNTING_HOLE]  177.8,0 90 top
U$16  141.38,10.62 0 top
U$18  93.98,4.83 0 top
U$20  PCB_MOUNTING_HOLE  [PCB_MOUNTING_HOLE]  177.8,78.11 90 top
U$21  [ICON_USA]  175.01,22.48 270 top
U$22  [ICON_MINUS]  23.75,10.16 180 top
U$23  PCB_MOUNTING_HOLE  [PCB_MOUNTING_HOLE]  93.34,78.11 90 top
U$24  [ICON_PLUS]  28.77,10.16 90 top
U$25  PCB_MOUNTING_HOLE  [PCB_MOUNTING_HOLE]  8.89,78.11 90 top
U$26  PCB_MOUNTING_HOLE  [PCB_MOUNTING_HOLE]  177.8,78.11 90 top
U$27  [VISION_REF15]  2.54,76.2 270 top
U$28  [VISION_REF10]  175.9,76.2 270 top
X1  38.61,5.08 180 top
X2  26.23,4.06 0 top
X3  52.7,5.08 180 top
X4  151.76,74.93 180 top
X5  136.53,74.93 180 top
X6  121.28,74.93 180 top
X7  106.05,74.93 180 top
X8  67.31,74.93 180 top
X9  52.07,74.93 180 top
X10  36.83,74.93 180 top
X11  21.59,74.93 180 top

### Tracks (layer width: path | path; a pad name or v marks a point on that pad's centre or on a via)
GND  (via drill 0.5, 0.6)
  Top 0.254: IC3.11 63.16,23.66 63.5,24 63.5,24.77 62.87,25.4 61.59,25.4 60.96,24.77 60.96,23.37 61.34,22.99 61.84,22.99 IC3.9
  Top 0.406: 34.8,12.38 X1.4
  Top 0.61: C4.1 C2.1 C3.1 | C5.1 87.22,14.84 | C7.1 C6.1 C8.1 66.04,17.14 67.31,17.14 68.58,15.88 | C9.1 67.54,14.84 68.58,15.88 | 68.58,15.88 U$6.GND
  Top 0.813: X3.1 56.52,12.06
  other vias: 5.71,15.11 6.03,18.1 156.84,38.1 73.03,25.4 139.06,38.1 118.11,36.2 105.66,9.27 146.69,5.08 116.2,3.81 152.4,5.08 158.12,5.08 140.97,5.08 135.25,5.08 129.54,5.08 123.83,5.08 110.49,24.13 77.09,23.11 30.48,34.92 54.61,38.1 72.39,38.1 147.96,30.48 136.53,17.14 87.25,21.34 87.63,50.8 80.64,38.1
  pour Top (isolate 0.305): 8.89,-1.27 8.89,8.89 -2.54,8.89 -2.54,78.11 8.89,78.11 8.89,41.91 84.45,41.91 84.45,78.11 93.34,78.11 93.34,41.91 168.91,41.91 168.91,78.11 179.07,78.11 179.71,78.74 179.71,8.89 168.91,8.89 168.91,-1.27 168.28,-1.91 8.89,-1.91
  pour Bottom (isolate 0.305): 8.89,-1.91 8.89,8.89 -10.16,8.89 -10.16,78.11 8.89,78.11 8.89,41.91 84.45,41.91 84.45,78.11 93.34,78.11 93.34,41.91 168.91,41.91 168.91,78.11 179.07,78.11 179.71,78.74 179.71,8.89 168.91,8.89 168.91,-1.27 168.28,-1.91
GP4
  Top 0.305: RN6.5 110.42,10.09 111.12,10.79 111.12,15.24 112.39,16.51 115.15,16.51 IC4.14 116.91,16.58 118.11,17.78 119.18,17.78 IC5.4
GP6
  Top 0.305: RN6.7 108.82,11.03 109.86,12.06 109.86,16.51 112.39,19.05 115.15,19.05 IC4.16 116.91,19.12 118.11,20.32 119.18,20.32 IC5.2
I2C_SCL  (via drill 0.9)
  Top 0.254: v48.9,27.3 50.16,26.04 64.77,26.04 65.15,25.65 65.15,23.05 | 65.15,23.05 IC3.14 | 65.15,23.05 65.15,22.35 66.04,21.46 67.69,21.46 69.22,19.94 71.63,19.94 73.28,21.59 83.95,21.59 84.58,22.23 104.14,22.23 104.78,21.59 105.89,21.59 IC4.1
  Top 0.406: RNE.4 44.51,14.68 42.55,12.7
  Top 0.813: X3.4 48.9,7.62 42.55,7.62 42.55,12.7 X1.1
  Bottom 0.813: v48.9,27.3 X3.4 48.9,12.06
  Bottom 1.016: 48.9,11.43 X3.4
I2C_SDA  (via drill 0.6, 0.9)
  Top 0.254: RNE.3 45.36,15.47 45.72,15.11 v45.72,10.16 | v51.44,27.3 52.32,26.54 65.15,26.54 65.79,25.91 65.79,23.04 | 65.79,23.04 IC3.15 | 65.79,23.04 65.79,22.48 66.29,21.97 67.94,21.97 69.47,20.45 71.37,20.45 73.03,22.1 83.69,22.1 84.33,22.73 107.7,22.73 108.08,22.35 108.08,20.7 107.82,20.45 IC4.2
  Top 0.61: X3.3 51.44,12.06 | X1.2 39.88,12.38
  Bottom 0.813: 39.88,12.38 39.88,11.56 41.27,10.16 v45.72,10.16 50.8,10.16 51.44,10.79 | X3.3 v51.44,27.3
  Bottom 1.016: 39.88,12.38 X1.2 | 51.44,10.79 51.44,12.06 X3.3
N$1  (via drill 0.6)
  Top 0.813: CB1.2 CA1.2 1.99,15.96 2.54,16.51 IC1.8 v5.46,16.51
  Top 1.27: v12.7,16.51 13.34,17.14 22.23,17.14 23.24,18.16 26.04,18.16 27.18,17.02 27.18,14.22 28.07,13.34 BRA1.+
  Bottom 1.27: v12.7,16.51 v5.46,16.51
N$2
  Top 0.305: RNB.3 21.4,18.95 21.4,18.7 21.12,18.41 13.78,18.41 13.45,18.74 POWER.A
N$3
  Top 0.254: 22.23,18.95 22.23,19.74 21.9,20.07 16.94,20.07
  Top 0.305: RNB.4 22.23,18.95 | 16.94,20.07 I2C.A
N$4  (via drill 0.6)
  Top 0.254: RNE.5 46.52,12.6 v46.67,12.57
  Bottom 0.254: U$3.A1 6.99,26.67 32.07,26.67 38.73,20 40.96,20 41.85,19.11 44.51,19.11 44.7,19.3 46.67,19.3 46.99,18.99 46.99,17.78 46.8,17.59 46.8,12.7 v46.67,12.57
N$5  (via drill 0.6)
  Top 0.254: RNE.6 46.12,15.47 45.72,15.88 v45.72,18.41
  Bottom 0.254: v45.72,18.41 41.53,18.41 41.02,18.92 38.54,18.92 31.5,25.97 8.95,25.97 6.35,23.5 U$3.B1
N$6
  Top 0.406: IC3.5 63.81,30.79 65.41,32.38 76.83,32.38 77.47,33.02 77.47,34.77 CD6.1 77.88,35.92 76.83,36.96 ACS5.7
N$7
  Top 1.016: ACS1.1 162.56,48.26 161.93,48.9 160.66,50.16 160.66,66.04 156.21,70.48 156.21,73.02 X4.2 152.4,73.61 152.4,71.12 155.57,67.94 155.57,53.98 161.29,48.26 ACS1.2
  Top 1.27: 161.93,48.9 161.93,52.7 161.29,53.34 161.29,50.16
  Top 1.778: 154.31,74.88 X4.2
N$8
  Top 1.016: 21.59,43.18 21.59,45.72
N$9
  Top 0.406: IC3.1 66.41,29.58 66.67,29.84 78.11,29.84 79.38,31.11 109.22,31.11 109.86,31.75 161.93,31.75 162.56,32.38 162.56,35.08 CD8.1 162.33,35.79 161.29,36.83 ACS1.7
N$10
  Top 0.406: IC3.2 65.76,29.82 66.42,30.48 77.72,30.48 78.99,31.75 108.84,31.75 109.47,32.38 143.64,32.38 144.53,33.27 144.53,35.16 CD4.1 144.55,35.79 143.64,36.7 143.64,37.9 ACS2.7
N$11
  Top 0.406: IC3.3 65.11,30.18 66.04,31.11 77.47,31.11 78.74,32.38 108.58,32.38 109.22,33.02 125.6,33.02 126.75,34.16 126.75,35.16 CD7.1 126.77,35.66 125.73,36.7 ACS3.7
N$12
  Top 0.406: IC3.4 64.46,30.55 65.66,31.75 77.22,31.75 78.49,33.02 108.33,33.02 108.84,33.53 108.84,35.03 CD3.1 108.99,35.79 107.95,36.83 ACS4.7
N$13
  Top 1.016: ACS2.2 143.51,48.26 137.79,53.98 137.79,73.61 X5.2 140.34,73.66 140.97,73.03 140.97,66.04 142.88,64.14 142.88,53.34 142.88,52.07 142.88,50.16 144.15,48.9 144.78,48.26 ACS2.1
  Top 1.27: 144.15,48.9 144.15,50.8 | 144.15,50.8 142.88,52.07 142.88,50.8 143.51,50.16 | 144.15,50.8 144.15,52.7 143.51,53.34 142.88,53.34
N$14
  Top 0.406: ACS6.7 59.05,36.83 60.33,35.56 60.33,35.41 CD2.1 60.09,33.76 63.12,30.73 63.12,29.1 IC3.6
N$15
  Top 0.406: 41.27,38.1 ACS7.7 41.27,36.83 42.29,35.81 42.29,35.2 CD5.1 42.31,32.62 43.18,31.75 61.21,31.75 62.48,30.48 62.48,29.09 IC3.7
N$16
  Top 1.016: 24.13,43.18 24.13,48.26 22.23,50.16 22.23,53.34 22.23,67.94 25.4,71.12 25.4,73.03 24.13,74.3 22.86,73.03 22.86,69.85 19.68,66.67 19.68,52.7 20.32,52.07 | 20.32,52.07 21.59,50.8 21.59,53.98 21.59,67.94 20.32,66.67 20.32,52.07 | 20.32,52.07 20.95,52.07 20.95,67.31 23.5,69.85 | 24.13,70.48 24.77,71.12 24.77,73.03 24.13,73.66 24.13,70.48 | 24.13,70.48 23.5,69.85 | 23.5,69.85 23.5,73.03
  Top 1.27: 24.13,48.26 24.13,52.7 23.5,53.34 22.23,53.34 22.23,52.7 23.5,51.44 | 23.5,51.44 23.5,50.16 | 23.5,51.44 23.5,52.07 21.59,53.98
N$17  (via drill 0.5)
  Top 0.254: IC3.12 63.81,21.9 v63.5,21.59 | v66.04,8.26 66.04,6.6
  Top 0.406: U$4.A1 73.66,9.27 70.99,6.6 66.04,6.6 65.13,6.6 RN1.4
  Bottom 0.254: v63.5,21.59 63.5,9.53 64.14,8.89 65.41,8.89 v66.04,8.26
N$18  (via drill 0.5)
  Top 0.254: IC3.13 64.46,21.9 v64.77,21.59 | v64.77,10.16 64.77,7.87 64.26,7.37 64.26,5.84 64.39,5.71 65.04,5.71 RN1.3 | U$4.A2 73.03,6.99 71.75,5.71 65.08,5.71
  Top 0.406: 65.08,5.71 RN1.3
  Bottom 0.254: v64.77,21.59 v64.77,10.16
N$20
  Top 1.016: 39.37,46.35 39.37,43.18
N$21
  Top 1.016: ACS4.2 107.95,48.26 103.5,52.7 103.5,66.67 106.68,69.85 106.68,72.98 X7.2 109.86,73.66 109.86,69.85 107.31,67.31 107.31,50.16 108.58,48.9 109.22,48.26 ACS4.1
  Top 1.27: 108.58,48.9 108.58,52.7 107.95,53.34 107.95,50.16
N$22
  Top 1.016: ACS4.4 105.41,46.99 K5_B2.COM 106.68,45.72 ACS4.3
N$23
  Top 1.016: ACS5.2 76.83,48.26 71.75,53.34 71.75,67.31 67.94,71.12 67.94,72.98 X8.2 71.75,73.02 71.75,70.48 76.2,66.04 76.2,50.16 77.47,48.9 78.11,48.26 ACS5.1 | 75.56,50.16 75.56,50.8 72.39,53.98 72.39,67.94 68.58,71.75 68.58,73.03 69.85,74.3 71.12,73.03 71.12,70.48 75.56,66.04 75.56,53.34 75.56,51.44 73.03,53.98 73.03,67.31 | 73.03,67.94 73.03,67.31 | 73.03,67.31 74.93,65.41 74.93,53.34 | 74.93,52.7 74.93,53.34 | 74.93,53.34 73.66,54.61 73.66,66.04 74.3,65.41 74.3,54.61
  Top 1.27: 77.47,48.9 77.47,52.7 76.83,53.34 75.56,53.34 76.83,52.07 76.83,50.16
N$24
  Top 1.016: 41.91,48.26 41.91,43.18 | ACS7.2 41.27,48.26 36.2,53.34 36.2,65.41 37.47,66.67 37.47,72.98 X10.2 40.64,73.66 40.64,53.34 40.64,50.16 42.55,48.26 ACS7.1
  Top 1.27: 41.91,48.26 41.91,52.7 41.27,53.34 40.64,53.34 40.64,51.44 41.27,50.8
N$25
  Top 1.016: ACS6.2 59.05,48.26 53.34,53.98 53.34,73.61 X9.2 55.88,73.66 55.88,66.67 58.42,64.14 58.42,50.16 59.69,48.9 60.33,48.26 ACS6.1 | 53.98,73.66 53.98,53.98 57.78,50.16 57.78,63.5 54.61,66.67 54.61,74.3 55.24,73.66 55.24,53.98 | 55.24,53.34 55.24,53.98 | 55.24,53.98 54.61,54.61 54.61,66.04 57.15,63.5 57.15,53.34 57.15,51.44
  Top 1.27: 59.69,48.9 59.69,52.7 59.05,53.34 57.78,53.34 | 57.15,53.34 57.78,53.34 | 57.78,53.34 59.05,52.07 59.05,50.16
N$26
  Top 1.016: 40.01,50.16 40.01,73.66 39.37,74.3 38.1,73.03 38.1,52.07 39.37,50.8 39.37,73.66 38.73,73.03 38.73,52.07 37.47,53.34 37.47,65.41 | 37.47,66.04 37.47,65.41 | 37.47,65.41 36.83,64.77 36.83,53.34
N$29
  Top 1.016: ACS8.2 23.5,48.26 19.05,52.7 19.05,66.67 22.23,69.85 22.23,72.98 X11.2 26.04,73.02 26.04,70.48 22.86,67.31 22.86,50.16 24.77,48.26 ACS8.1
N$30
  Top 1.016: 56.52,52.07 56.52,63.5 55.88,64.14
N$31  (via drill 0.5)
  Top 1.016: C2.2 C4.2 87.55,19.91 U$5.IN 90.81,19.66 v90.81,20.95 | BRA3.+ v88.9,5.71
  Bottom 1.016: v88.9,5.71 90.17,5.71 90.81,6.35 v90.81,20.95
N$32  (via drill 0.5)
  Top 1.016: C6.2 C8.2 67.86,19.91 U$6.IN 71.5,18.16 72.39,19.05 72.39,19.43 73.03,20.07 78.99,20.07 80.01,19.05 v80.01,12.06 | v82.55,5.71 BRA4.+
  Bottom 1.016: v80.01,12.06 80.01,6.99 81.28,5.71 v82.55,5.71
N$33
  Top 0.254: CE1.1 160,38 ACS1.6
N$34
  Top 0.254: CE2.1 142.22,38 ACS2.6
N$35
  Top 0.254: CE3.1 124.44,38 ACS3.6
N$36
  Top 0.254: CE4.1 106.66,38 ACS4.6
N$37
  Top 0.406: IC3.8 61.86,30.21 60.96,31.11 25.4,31.11 24.77,31.75 24.77,34.95 CD1.1 24.54,35.79 23.5,36.83 ACS8.7
N$38
  Top 0.254: CE5.1 75.54,38 ACS5.6
N$39
  Top 0.254: CE6.1 57.76,38 ACS6.6
N$40
  Top 0.254: CE7.1 40.01,35.18 ACS7.6
N$41
  Top 0.254: CE8.1 22.23,35.18 ACS8.6
N$42
  Top 1.016: ACS1.3 160.02,45.72 K8_B2.COM 158.75,46.99 ACS1.4
N$43
  Top 1.016: K8_B2.NC 152.15,66.29 149.22,69.22 149.22,74.88 X4.3
N$44
  Top 1.016: K8_B2.NO 164.08,67.06 159.38,71.75 159.38,74.88 X4.1
N$45
  Top 1.016: K7_B2.NO 146.3,65.79 144.15,67.94 144.15,74.88 X5.1
N$46
  Top 1.016: K6_B2.NO 128.52,74.5 X6.1
N$47  (via drill 0.5)
  Top 0.254: RN2.2 101.96,17.13 101.73,16.89 101.73,15.62 101.35,15.24 v100.33,15.24
  Top 0.406: IC4.5 104.01,16.64 103.5,17.14 102.55,17.14 RN2.2
  Bottom 0.254: v100.33,15.24 100.97,14.61 100.97,10.54 100.33,9.91 U$18.B1
N$48  (via drill 0.5)
  Top 0.254: v100.97,20.32 101.73,19.56 101.73,18.16 101.98,17.91 102.51,17.91 RN2.3
  Top 0.406: IC4.4 102.55,17.91 RN2.3
  Bottom 0.406: U$18.B2 101.35,7.37 101.6,7.62 101.6,19.05 100.97,19.68 v100.97,20.32
N$49  (via drill 0.5)
  Top 0.406: IC4.3 102.98,19.18 RN2.4 102.49,18.76 v102.49,20.32
  Bottom 0.406: U$18.B3 102.23,4.83 102.49,5.08 v102.49,20.32
N$50
  Top 0.305: RN5.7 112.5,13.44 113.03,13.97 115.15,13.97 IC4.12 116.91,14.04 118.11,15.24 119.18,15.24 IC5.6
N$51
  Top 0.305: RN5.6 113.3,12.34 113.67,12.7 115.15,12.7 IC4.11 116.91,12.77 118.11,13.97 119.18,13.97 IC5.7
N$52
  Top 0.254: 115.15,11.43 IC4.10
  Top 0.305: RN5.5 114.1,10.38 IC4.10 116.91,11.5 118.11,12.7 119.18,12.7 IC5.8
N$53
  Top 0.406: RN3.1 134.78,9.05 133.99,8.26 120.4,8.26 119.89,7.75 119.89,5.09 R1.C
N$54
  Top 0.406: RN3.2 135.66,14.21 135.89,13.97 135.89,8.89 134.62,7.62 125.98,7.62 125.6,7.24 125.6,5.09 R2.C
N$55
  Top 0.406: RN3.3 136.12,15.01 136.53,14.61 136.53,8.26 135.25,6.99 131.95,6.99 131.32,6.35 131.32,5.09 R3.C
N$56
  Top 0.406: RN3.4 136.59,15.8 137.16,15.24 137.16,5.84 137.03,5.71 137.03,5.09 R4.C
N$57
  Top 0.406: RN4.8 138.5,20.89 139.7,19.68 139.7,10.16 140.97,8.89 159.38,8.89 160.02,8.26 160.02,5.2 R8.C
N$76
  Top 2.54: 74.95,74.91 74.95,71.73 79.38,67.31 79.38,62.1 79.63,61.85
N$77
  Top 2.54: 64.79,74.91 64.79,69.83 67.31,67.31 67.31,62.23 67.69,61.85
N$79
  Top 2.54: 59.71,74.91 59.71,67.29 61.59,65.41 61.59,62.1 61.85,61.85
N$80
  Top 2.54: 49.55,74.91 49.55,62.21 49.91,61.85
N$81
  Top 0.406: RN4.7 138.03,20.09 139.06,19.05 139.06,9.53 140.34,8.26 153.67,8.26 154.31,7.62 154.31,5.2 R7.C
N$82
  Top 0.406: RN4.6 137.56,19.29 138.43,18.41 138.43,8.89 139.7,7.62 147.96,7.62 148.34,7.24 148.34,5.22 R6.C
N$83
  Top 0.406: RN4.5 137.09,18.48 137.79,17.78 137.79,8.26 139.06,6.99 142.24,6.99 142.88,6.35 142.88,5.2 R5.C
N$85
  Top 2.54: 44.47,74.91 44.47,62.25 44.07,61.85
N$86
  Top 2.54: 34.31,74.91 34.31,67.97 32.38,66.04 32.38,62.1 32.13,61.85
N$88
  Top 2.54: 29.23,74.91 29.23,69.24 26.67,66.67 26.67,62.23 26.29,61.85
N$89
  Top 0.305: RN5.8 111.7,14.55 112.39,15.24 115.15,15.24 IC4.13 116.91,15.31 118.11,16.51 119.18,16.51 IC5.5
N$90
  Top 2.54: 19.07,74.91 19.07,71.14 14.61,66.67 14.61,62.1 14.35,61.85
N$93
  Top 0.305: RN6.6 109.62,10.56 110.49,11.43 110.49,15.88 112.39,17.78 115.15,17.78 IC4.15 116.91,17.85 118.11,19.05 119.18,19.05 IC5.3
N$94
  Top 0.305: RN6.8 108.02,11.5 109.22,12.7 109.22,17.14 112.39,20.32 115.12,20.32 IC4.17 116.94,20.42 118.11,21.59 119.18,21.59 IC5.1
N$95
  Bottom 2.54: 14.35,61.85 14.35,66.42 19.05,71.12 19.05,74.88 19.07,74.91
N$96
  Bottom 2.54: 26.29,61.85 26.29,65.66 29.21,68.58 29.21,74.88 29.23,74.91
N$97
  Bottom 2.54: 44.07,61.85 44.07,64.39 44.45,64.77 44.45,74.88 44.47,74.91
N$98
  Bottom 2.54: 61.85,61.85 61.85,65.15 59.69,67.31 59.69,74.88 59.71,74.91
N$99
  Bottom 2.54: 32.13,61.85 32.13,65.15 34.29,67.31 34.29,74.88 34.31,74.91
N$101
  Bottom 2.54: 49.91,61.85 49.91,64.39 49.53,64.77 49.53,73.61 49.55,74.91
N$102
  Top 2.54: 49.53,64.14 49.53,74.93 50.16,74.93 50.16,64.14 | 49.53,64.14 50.16,64.14 | 50.16,64.14 50.16,63.5 | 50.16,63.5 50.16,61.59 49.53,61.59 49.53,62.23 | 49.53,62.23 49.53,63.5 | 49.53,64.14 49.53,63.5 | 49.53,63.5 50.16,63.5 | 49.53,62.23 50.8,62.23 | 50.8,62.23 50.8,74.93 48.26,74.93 48.26,60.96 50.8,60.96 50.8,62.23
N$103
  Bottom 2.54: 54.61,74.88 54.63,74.91
N$106
  Top 2.54: 59.05,67.94 59.05,74.93 60.33,74.93 60.33,68.58 62.87,66.04 62.87,60.96 60.96,60.96 60.96,65.41 | 59.05,67.94 60.96,66.04 60.96,65.41 | 59.05,67.94 59.05,67.31 60.96,65.41
N$107
  Top 2.54: 66.67,60.96 66.67,66.67 64.14,69.22 64.14,74.93 65.41,74.93 65.41,69.85 68.58,66.67 68.58,60.96 66.67,60.96
N$109
  Top 2.54: 74.3,74.93 74.3,71.75 78.74,67.31 78.74,60.96 80.64,60.96 80.64,67.31 75.56,72.39 75.56,74.93 74.3,74.93
N$110
  Top 2.54: 45.09,74.93 45.09,60.96 43.18,60.96 43.18,74.93 45.09,74.93
N$112
  Top 2.54: 34.92,74.93 34.92,67.94 33.66,66.67 33.66,60.96 31.11,60.96 31.11,66.04 33.66,68.58 33.66,74.93 34.92,74.93
N$113
  Top 2.54: 29.21,74.93 29.84,74.93 29.84,69.22 27.3,66.67 27.3,60.96 25.4,60.96 25.4,66.04 28.57,69.22 | 29.21,69.85 29.21,74.93 | 29.21,74.93 28.57,74.93 28.57,68.58
N$115
  Top 2.54: 19.68,74.93 19.68,71.12 15.24,66.67 15.24,60.96 13.34,60.96 13.34,66.04 18.41,71.12 18.41,74.93 19.68,74.93
N$116
  Bottom 2.54: 19.05,74.93 18.41,74.93 18.41,71.12 13.34,66.04 13.34,60.96 15.24,60.96 15.24,66.67 19.68,71.12 19.68,74.93
N$118
  Bottom 2.54: 28.57,74.93 28.57,69.22 25.4,66.04 25.4,60.96 27.3,60.96 27.3,66.67 29.84,69.22 29.84,74.93 28.57,74.93
N$119
  Bottom 2.54: 33.66,74.93 33.66,68.58 31.11,66.04 31.11,60.96 33.66,60.96 33.66,66.67 34.92,67.94 34.92,74.93 33.66,74.93
N$121
  Bottom 2.54: 45.09,74.93 43.18,74.93 43.18,60.96 45.09,60.96 45.09,74.93
N$122
  Bottom 2.54: 48.26,74.93 48.26,60.96 50.8,60.96 50.8,74.93 48.26,74.93
N$124
  Bottom 2.54: 59.05,74.93 59.05,67.31 60.96,65.41 60.96,60.96 62.87,60.96 62.87,66.04 60.33,68.58 60.33,74.93 59.05,74.93
N$125
  Bottom 2.54: 67.69,61.85 67.69,65.66 66.67,66.67 | 66.67,66.67 64.77,68.58 | 64.77,68.58 64.77,74.88 64.79,74.91 | 64.77,68.58 64.14,69.22 64.14,74.93 65.41,74.93 65.41,69.85 68.58,66.67 68.58,60.96 66.67,60.96 66.67,66.67
N$127
  Bottom 2.54: 79.63,61.85 79.63,66.42 78.74,67.31 | 78.74,67.31 74.93,71.12 | 74.93,71.12 74.93,74.88 74.95,74.91 | 74.93,71.12 74.3,71.75 74.3,74.93 75.56,74.93 75.56,72.39 80.64,67.31 80.64,60.96 78.74,60.96 78.74,67.31
N$137
  Top 1.016: K7_B2.NC 134.37,74.55 X5.3
N$138
  Top 1.016: ACS2.4 140.97,46.99 K7_B2.COM 141.6,46.35 | ACS2.3 142.24,45.72 141.6,46.35 | 141.6,46.35 141.6,43.18
N$139
  Top 1.016: K6_B2.NC 116.59,66.42 118.75,68.58 118.75,74.88 X6.3
N$140
  Top 1.016: ACS3.4 123.19,46.99 K6_B2.COM 124.46,45.72 ACS3.3
N$141
  Top 1.016: K5_B2.NC 98.81,67.06 103.5,71.75 103.5,74.88 X7.3
N$142
  Top 1.016: 55.88,63.5 55.88,52.7
N$143
  Top 1.016: K5_B2.NO 110.74,66.29 113.67,69.22 113.67,74.88 X7.1
N$144
  Top 1.016: K4_B2.NO 79.63,67.06 74.93,71.75 74.93,74.88 X8.1
N$145
  Top 1.016: K4_B2.NC 67.69,66.29 64.77,69.22 64.77,74.88 X8.3
N$146
  Top 1.016: ACS5.4 74.3,46.99 K4_B2.COM 74.3,47.62 75.56,46.35 ACS5.3
N$147
  Top 1.016: K3_B2.NO 61.85,65.79 59.69,67.94 59.69,74.88 X9.1
N$148
  Top 1.016: K3_B2.NC 49.91,74.55 X9.3
N$149
  Top 1.016: ACS6.4 56.52,46.99 K3_B2.COM 57.78,45.72 ACS6.3
N$150
  Top 1.016: K2_B2.NO 44.07,74.5 X10.1
N$151
  Top 1.016: K2_B2.NC 32.13,66.42 34.29,68.58 34.29,74.88 X10.3
N$152
  Top 1.016: ACS7.4 38.73,46.99 K2_B2.COM 38.1,48.26 40.01,46.35 ACS7.3
N$153
  Top 1.016: K1_B2.NO 26.29,66.29 29.21,69.22 29.21,74.88 X11.1
N$154
  Top 1.016: K1_B2.NC 14.35,66.42 19.05,71.12 19.05,74.88 X11.3
N$155
  Top 1.016: ACS8.4 20.95,46.99 K1_B2.COM 22.23,45.72 ACS8.3
N$156
  Top 1.016: 57.15,45.72 57.15,43.18
N$157
  Top 1.016: 59.69,48.26 59.69,43.18
N$158
  Top 1.016: 74.93,46.35 74.93,43.18
N$159
  Top 1.016: 77.47,48.26 77.47,45.09 77.47,43.81 77.47,43.18
N$161
  Top 1.016: 70.48,70.48 70.48,72.39 69.85,73.03 69.22,72.39 69.85,71.75 69.85,71.12
N$162
  Top 1.016: 106.05,45.72 106.05,43.18
N$163
  Top 1.016: 108.58,48.26 108.58,43.18
N$164
  Top 1.016: 106.68,50.16 106.68,67.94 109.22,70.48 109.22,73.03 108.58,73.66 107.95,73.03 | 107.95,73.03 107.31,72.39 107.31,69.85 108.58,71.12 108.58,72.39 107.95,73.03 | 107.95,73.03 107.95,69.85 104.14,66.04 104.14,53.34 106.05,51.44 106.05,52.07 106.05,66.67 | 106.05,67.31 106.05,66.67 | 106.05,66.67 104.78,65.41 104.78,53.98 105.41,53.34 105.41,65.41
  Top 1.27: 106.05,50.8 106.05,52.07
N$165
  Top 1.016: 123.83,45.72 123.83,43.18
N$166
  Top 1.016: 126.36,48.26 126.36,43.18 | ACS3.2 125.73,48.26 121.28,52.7 121.28,66.67 121.92,67.31 121.92,72.98 X6.2 125.09,73.66 125.09,51.44 125.09,50.16 127,48.26 ACS3.1
  Top 1.27: 126.36,48.26 126.36,50.16 | 126.36,50.16 125.09,51.44 | 124.46,50.8 125.09,50.16 | 126.36,50.16 126.36,52.7 125.73,53.34 125.73,51.44
N$167
  Top 1.016: 124.46,50.16 122.56,52.07 | 122.56,52.07 121.92,52.7 121.92,66.04 123.19,67.31 123.19,74.3 123.83,74.93 123.83,66.67 | 123.83,66.67 123.83,52.07 124.46,51.44 124.46,73.66 | 122.56,73.03 122.56,52.07 | 122.56,52.07 123.19,52.7 123.19,66.04 123.83,66.67
N$168
  Top 1.016: 144.15,48.26 144.15,43.18
N$170
  Top 1.016: 141.6,64.14 140.97,64.14 139.06,66.04 139.06,73.03 139.7,73.03 | 142.24,50.16 138.43,53.98 138.43,73.03 139.06,73.66 139.7,73.03 | 139.7,73.03 140.34,72.39 140.34,52.7 140.97,52.07 | 140.97,52.07 142.24,50.8 142.24,64.14 140.97,65.41 140.97,52.07 | 140.97,52.07 141.6,52.7 141.6,63.5 | 139.7,73.03 139.7,53.98 | 139.7,53.34 139.7,53.98 | 139.7,53.98 139.06,54.61 139.06,65.41
N$171
  Top 1.016: 159.38,45.72 159.38,43.18
N$172
  Top 1.016: 161.93,48.26 161.93,43.18
N$173
  Top 1.016: 155.57,70.48 155.57,73.03 154.31,74.3 153.67,73.66 153.03,73.66 153.03,71.75 156.21,68.58 156.21,53.98 160.02,50.16 160.02,50.8 | 155.57,70.48 155.57,69.85 160.02,65.41 160.02,51.44 | 155.57,70.48 153.67,72.39 153.67,73.03 154.31,73.66 154.94,73.03 154.94,72.39 | 154.94,71.75 154.94,72.39 | 154.94,72.39 154.31,73.03
N$174
  Top 1.016: 159.38,51.44 159.38,65.41 156.84,67.94 156.84,53.98 157.48,53.34 | 158.12,52.7 158.75,52.07 158.75,65.41 157.48,66.67 157.48,53.34 | 157.48,53.34 158.12,52.7 | 158.12,52.7 158.12,65.41
N$305
  Top 2.54: 149.25,74.91 149.25,69.19 151.76,66.67 151.76,62.23 152.15,61.85
N$306
  Top 2.54: 159.41,74.91 159.41,71.73 163.83,67.31 163.83,62.1 164.08,61.85
N$307
  Top 2.54: 144.17,74.91 144.17,67.92 146.05,66.04 146.05,62.1 146.3,61.85
N$308
  Top 2.54: 128.93,74.91 128.93,62.25 128.52,61.85
N$309
  Top 2.54: 134.01,74.91 134.01,62.21 134.37,61.85
N$311
  Top 2.54: 118.77,74.91 118.77,67.97 116.84,66.04 116.84,62.1 116.59,61.85
N$313
  Top 2.54: 103.53,74.91 103.53,71.14 98.42,66.04 98.42,62.23 98.81,61.85
N$315
  Top 2.54: 113.69,74.91 113.69,69.24 110.49,66.04 110.49,62.1 110.74,61.85
N$360
  Top 2.54: 113.69,74.91 113.69,69.24 111.12,66.67 111.12,62.23 110.74,61.85
N$361
  Top 2.54: 103.53,74.91 103.53,71.14 99.06,66.67 99.06,62.1 98.81,61.85
N$363
  Top 2.54: 128.93,74.91 128.93,62.25 128.52,61.85
N$364
  Top 2.54: 118.77,74.91 118.77,67.97 116.84,66.04 116.84,62.1 116.59,61.85
N$366
  Top 2.54: 144.17,74.91 144.17,67.29 146.05,65.41 146.05,62.1 146.3,61.85
N$367
  Top 2.54: 134.01,74.91 134.01,62.21 134.37,61.85
N$369
  Top 2.54: 159.41,74.91 159.41,71.73 163.83,67.31 163.83,62.1 164.08,61.85
N$370
  Top 2.54: 149.25,74.91 149.25,69.83 152.4,66.67 152.4,62.1 152.15,61.85
N$373
  Bottom 2.54: 98.81,61.85 98.81,66.42 103.5,71.12 103.5,74.88 103.53,74.91
N$374
  Bottom 2.54: 110.74,61.85 110.74,65.66 113.67,68.58 113.67,74.88 113.69,74.91
N$375
  Bottom 2.54: 128.52,61.85 128.52,64.39 128.91,64.77 128.91,74.88 128.93,74.91
N$376
  Bottom 2.54: 146.3,61.85 146.3,65.15 144.15,67.31 144.15,74.88 144.17,74.91
N$377
  Bottom 2.54: 116.59,61.85 116.59,65.15 118.75,67.31 118.75,74.88 118.77,74.91
N$379
  Bottom 2.54: 134.37,61.85 134.37,64.39 133.99,64.77 133.99,73.61 134.01,74.91
N$380
  Top 2.54: 133.99,64.14 133.99,74.93 134.62,74.93 134.62,64.14 | 133.99,64.14 134.62,64.14 | 134.62,64.14 134.62,63.5 | 134.62,63.5 134.62,61.59 133.99,61.59 133.99,62.23 | 133.99,62.23 133.99,63.5 | 133.99,64.14 133.99,63.5 | 133.99,63.5 134.62,63.5 | 133.99,62.23 135.25,62.23 | 135.25,62.23 135.25,74.93 132.72,74.93 132.72,60.96 135.25,60.96 135.25,62.23
N$383
  Top 2.54: 143.51,74.93 143.51,67.31 145.41,65.41 145.41,60.96 147.32,60.96 147.32,66.04 144.78,68.58 144.78,74.93 143.51,74.93
N$384
  Top 2.54: 151.13,60.96 151.13,66.67 148.59,69.22 148.59,74.93 149.86,74.93 149.86,69.85 153.03,66.67 153.03,60.96 151.13,60.96
N$386
  Top 2.54: 158.75,74.93 158.75,71.75 163.19,67.31 163.19,60.96 165.1,60.96 165.1,67.31 160.02,72.39 160.02,74.93 158.75,74.93
N$387
  Top 2.54: 129.54,74.93 129.54,60.96 127.64,60.96 127.64,74.93 129.54,74.93
N$389
  Top 2.54: 119.38,74.93 119.38,67.94 118.11,66.67 118.11,60.96 115.57,60.96 115.57,66.04 118.11,68.58 118.11,74.93 119.38,74.93
N$390
  Top 2.54: 113.67,74.93 114.3,74.93 114.3,69.22 111.76,66.67 111.76,60.96 109.86,60.96 109.86,66.04 113.03,69.22 | 113.67,69.85 113.67,74.93 | 113.67,74.93 113.03,74.93 113.03,68.58
N$392
  Top 2.54: 104.14,74.93 104.14,71.12 99.69,66.67 99.69,60.96 97.79,60.96 97.79,66.04 102.87,71.12 102.87,74.93 104.14,74.93
N$393
  Bottom 2.54: 103.5,74.93 102.87,74.93 102.87,71.12 97.79,66.04 97.79,60.96 99.69,60.96 99.69,66.67 104.14,71.12 104.14,74.93
N$395
  Bottom 2.54: 113.03,74.93 113.03,69.22 109.86,66.04 109.86,60.96 111.76,60.96 111.76,66.67 114.3,69.22 114.3,74.93 113.03,74.93
N$396
  Bottom 2.54: 118.11,74.93 118.11,68.58 115.57,66.04 115.57,60.96 118.11,60.96 118.11,66.67 119.38,67.94 119.38,74.93 118.11,74.93
N$398
  Bottom 2.54: 129.54,74.93 127.64,74.93 127.64,60.96 129.54,60.96 129.54,74.93
N$399
  Bottom 2.54: 132.72,74.93 132.72,60.96 135.25,60.96 135.25,74.93 132.72,74.93
N$401
  Bottom 2.54: 143.51,74.93 143.51,67.31 145.41,65.41 145.41,60.96 147.32,60.96 147.32,66.04 144.78,68.58 144.78,74.93 143.51,74.93
N$402
  Bottom 2.54: 152.15,61.85 152.15,65.66 151.13,66.67 | 151.13,66.67 149.22,68.58 | 149.22,68.58 149.22,74.88 149.25,74.91 | 149.22,68.58 148.59,69.22 148.59,74.93 149.86,74.93 149.86,69.85 153.03,66.67 153.03,60.96 151.13,60.96 151.13,66.67
N$404
  Bottom 2.54: 164.08,61.85 164.08,66.42 163.19,67.31 | 163.19,67.31 159.38,71.12 | 159.38,71.12 159.38,74.88 159.41,74.91 | 159.38,71.12 158.75,71.75 158.75,74.93 160.02,74.93 160.02,72.39 165.1,67.31 165.1,60.96 163.19,60.96 163.19,67.31
OC_R1  (via drill 0.5)
  Top 0.305: IC5.11 131.32,12.83 131.95,13.46 133.13,13.46 RN3.8
  Top 0.406: v127,12.7 128.98,12.7 IC5.11
  Bottom 0.406: K8_B2.C1 165.61,49.66 167,48.26 167,13.97 165.74,12.7 v127,12.7
OC_R2  (via drill 0.5)
  Top 0.305: IC5.12 131.44,14.1 131.57,14.22 133.17,14.22 RN3.7
  Top 0.406: v127,13.97 128.98,13.97 IC5.12
  Bottom 0.406: K7_B2.C1 147.83,49.66 149.22,48.26 149.22,15.24 147.96,13.97 v127,13.97
OC_R3  (via drill 0.5)
  Top 0.305: IC5.13 131.32,15.37 131.7,14.99 133.17,14.99 RN3.6
  Top 0.406: v127,15.24 128.98,15.24 IC5.13
  Bottom 0.406: K6_B2.C1 130.05,49.66 131.44,48.26 131.44,16.64 130.18,15.37 127.13,15.37 v127,15.24
OC_R4  (via drill 0.5)
  Top 0.305: IC5.14 131.32,16.64 132.08,15.88 133.12,15.88 RN3.5
  Top 0.406: v127,16.51 128.98,16.51 IC5.14
  Bottom 0.406: K5_B2.C1 112.27,49.66 113.67,48.26 113.67,42.55 115.57,40.64 129.54,40.64 130.18,40.01 130.18,17.7 IC5.14 127.13,16.64 v127,16.51
OC_R5  (via drill 0.5)
  Top 0.305: IC5.15 131.57,17.91 132.08,18.41 133.12,18.41 RN4.4
  Top 0.406: v127,17.78 128.98,17.78 IC5.15
  Bottom 0.406: K4_B2.C1 79.63,46.48 81.03,45.09 95.25,45.09 96.52,43.81 96.52,40.64 97.16,40.01 128.91,40.01 129.54,39.37 129.54,18.34 IC5.15 127.13,17.91 v127,17.78
OC_R6  (via drill 0.5)
  Top 0.305: IC5.16 133.08,19.18 RN4.3
  Top 0.406: v127,19.05 128.98,19.05 IC5.16
  Bottom 0.406: K3_B2.C1 64.01,49.66 64.77,48.9 64.77,46.35 66.67,44.45 94.61,44.45 95.89,43.18 95.89,40.01 96.52,39.37 128.27,39.37 128.91,38.73 128.91,19.68 128.27,19.05 v127,19.05
OC_R7  (via drill 0.5)
  Top 0.305: IC5.17 131.32,20.45 131.7,20.07 133.17,20.07 RN4.2
  Top 0.406: v127,20.32 128.98,20.32 IC5.17
  Bottom 0.406: K2_B2.C1 46.23,49.66 46.99,48.9 46.99,46.35 49.53,43.81 93.98,43.81 95.25,42.55 95.25,39.37 95.89,38.73 127.64,38.73 128.27,38.1 128.27,20.95 127.64,20.32 v127,20.32
OC_R8  (via drill 0.5)
  Top 0.305: IC5.18 131.19,21.72 132.08,20.83 133.13,20.83 RN4.1
  Top 0.406: v127,21.59 128.98,21.59 IC5.18
  Bottom 0.406: K1_B2.C1 28.45,49.66 29.21,48.9 29.21,46.35 32.38,43.18 93.34,43.18 94.61,41.91 94.61,38.73 95.25,38.1 126.36,38.1 127,37.47 v127,21.59
REG_5V  (via drill 0.5)
  Top 0.254: RNB.6 21.42,21.29 21.21,21.5 | 21.21,21.5 20.99,21.72 3.62,21.72 3.17,22.16 U$3.B2 | U$4.B2 U$4.B1 | v70.48,21.72 CA4.1 | U$2.O2 21.21,21.5 | 113.03,22.23 108.58,17.78 108.58,16 107.95,15.37 | IC3.16 66.41,23.86 v67.31,24.77 | v62.48,24.26 62.48,23.04 IC3.10
  Top 0.406: IC3.16 70.23,23.01 CA4.1 75.33,23.27 76.2,24.13 76.2,26.04 C1.+ | CB3.2 84.22,25.17 | IC4.18 113.54,21.72 113.03,22.23 v113.03,23.5 113.03,25.68 CB6.2 CA7.2 | 127,3.17 121.92,3.17 121.4,3.69 R1.A 121.4,6.87 v121.28,6.99 | 127,3.17 132.72,3.17 | 132.72,3.17 138.43,3.17 | 138.43,3.17 144.15,3.17 | 144.15,3.17 149.86,3.17 | 149.86,3.17 155.57,3.17 | 155.57,3.17 160.66,3.17 161.29,3.81 161.29,4.96 R8.A | R7.A 155.69,3.29 155.57,3.17 | R6.A 149.97,3.29 149.86,3.17 | R5.A 144.26,3.29 144.15,3.17 | R4.A 138.54,3.29 138.43,3.17 | R3.A 132.83,3.29 132.72,3.17 | R2.A 127.11,3.29 127,3.17 | 107.95,15.37 IC4.6 105.89,15.24 103.5,15.24 102.23,13.97 99.69,13.97 99.06,13.34 99.06,12.06 98.42,11.43 94.61,11.43 93.98,10.79 U$18.A1 U$18.A2 U$18.A3
  Top 0.762: 83.82,24.13 84.45,23.5 107.95,23.5 108.58,24.13 108.58,25.38
  Top 0.813: C1.+ 74.3,26.67 73.03,27.94 67.94,27.94 67.31,27.3 59.05,27.3 v57.78,28.57 | v20.32,28.57 20.32,27.3 21.21,26.42 U$2.O2
  Top 1.016: C1.+ 76.83,25.4 78.11,24.13 83.82,24.13 84.45,24.77 84.45,25.42 CB3.2 CA3.2 82.55,28.57 v81.92,29.21 | 108.58,25.38 CA7.2 | v87,41.91 87,46.35 90.55,49.91 90.55,56.01 C10.+
  Bottom 0.254: U$4.B1 76.2,10.79 75.56,11.43 71.12,11.43 70.48,12.06 v70.48,21.72 | v67.31,24.77 62.87,24.77 v62.48,24.26
  Bottom 0.406: v121.28,6.99 114.3,6.99 113.67,7.62 113.67,22.86 v113.03,23.5
  Bottom 0.635: v57.78,28.57 v20.32,28.57
  Bottom 0.813: U$3.B2 U$3.A2
  Bottom 1.016: v81.92,29.21 85.72,29.21 87,30.48 v87,41.91
REG_5V_A  (via drill 0.5)
  Top 0.406: ACS1.8 162.56,40.64 | ACS2.8 144.78,40.64 | ACS3.8 127,40.64 | ACS4.8 109.22,40.64
  Top 1.016: C3.2 C5.2 87.55,11.84 U$5.OUT 89.31,15.47 v88.9,15.88 | v89.53,40.64 109.22,40.64 127,40.64 144.78,40.64 162.56,40.64
  Bottom 1.016: v88.9,15.88 88.9,40.01 v89.53,40.64
REG_5V_B  (via drill 0.5)
  Top 0.406: ACS5.8 v78.11,40.64 | ACS6.8 v60.33,40.64 | ACS7.8 42.55,40.64 | ACS8.8 24.77,40.64
  Top 1.016: U$6.OUT 69.47,13.6 67.94,12.06 66.27,12.06 C9.2 C7.2 60.55,11.84 v60.33,12.06 | 24.77,40.64 42.55,40.64 v48.26,40.64 v78.11,40.64
  Bottom 1.143: 58.42,29.84 52.7,29.84
  Bottom 1.27: v60.33,12.06 60.33,27.94 58.42,29.84 | 52.7,29.84 48.26,33.66 v48.26,40.64 | v78.11,40.64 v60.33,40.64
REG_5V_BUS  (via drill 0.5)
  Top 0.305: RNB.5 22.26,22.9 v22.23,22.99
  Top 0.61: X1.3 37.34,12.38 | X3.2 53.98,12.06
  Bottom 0.813: 37.34,12.38 37.34,11.43 37.34,11.05 39.37,8.89 52.7,8.89 53.98,10.16 53.98,12.06
  Bottom 1.016: v22.23,22.99 22.23,14.29 25.72,10.16 36.07,10.16 37.34,11.43 | 37.34,12.38 X1.3 | 53.98,12.06 X3.2
REG_5V_EXT  (via drill 0.5, 0.6)
  Top 0.813: CB2.2 CA2.2 9.76,15.64 8.89,16.51 | 8.89,16.51 IC1.1 | v10.92,17.91 10.92,17.27 10.16,16.51 8.89,16.51 | v17.14,24.13 U$2.O1
  Bottom 0.813: v17.14,24.13 v10.92,17.91
UNREG_12V  (via drill 0.5, 0.9)
  Top 0.406: v132.08,10.79 131.57,10.79 130.81,11.56 IC5.10
  Top 1.016: BRA4.~@2 BRA4.~@1 BRA3.~@2 BRA3.~@1 v62.87,2.54 | v58.42,9.53 58.42,23.5 57.78,24.13 43.81,24.13 43.18,24.77
  Top 1.27: C11.+ v154.94,10.79 | v43.18,27.3 25.4,27.3 20.95,31.75 16.64,31.75 14.35,34.04 K1_B2.C2
  Top 1.524: v43.18,27.3 43.18,24.77 43.18,24.13 41.91,22.86 36.7,22.86 32.89,19.05 32.89,9.08 29.11,5.3 28.57,4.76
  Top 2.286: BRA1.~@2 22.86,14.61 16.01,14.61
  Top 2.54: 16.01,14.61 U$1.TIP | X2.2 28.55,4.45 28.57,4.76 | BRA1.~@2 BRA1.~@1 24.13,12.45 28.57,8 28.57,5.84 29.11,5.3
  Bottom 1.016: v62.87,2.54 62.87,6.99 60.96,8.89 59.05,8.89 v58.42,9.53 | C11.+ 154.94,28.57 152.4,31.11 152.4,49.4 K8_B2.C2 152.15,51.05 150.5,52.7 134.62,52.7 | 134.62,52.7 116.84,52.7 | 116.84,52.7 99.06,52.7 | 99.06,52.7 67.94,52.7 | 67.94,52.7 50.16,52.7 | 50.16,52.7 32.38,52.7 | 32.38,52.7 14.61,52.7 13.97,52.07 13.97,50.04 K1_B2.C2 | K2_B2.C2 32.13,52.45 32.38,52.7 | K3_B2.C2 49.91,52.45 50.16,52.7 | K4_B2.C2 67.69,52.45 67.94,52.7 | K5_B2.C2 98.81,52.45 99.06,52.7 | K6_B2.C2 116.59,52.45 116.84,52.7 | K7_B2.C2 134.37,52.45 134.62,52.7
  Bottom 1.27: v154.94,10.79 v132.08,10.79

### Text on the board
tNames: IP- | IP+ | IP- | IP- | IP+ | IP- | IP- | IP+ | IP- | IP- | IP+ | IP- | IP- | IP+ | IP- | IP- | IP+ | IP- | IP- | IP+ | IP- | IP- | IP+ | IP- | NC | COM | NO | NC | COM | NO | NC | COM | NO | NC | COM | NO | NC | COM | NO | NC | COM | NO | NC | COM | NO | NC | COM | NO | 8 | 5 | 4 | 1 | Bank 1 | 8 | 8 | 7 | 7 | 6 | 6 | 5 | 5 | 4 | 4 | 3 | 3 | 2 | 2 | 1 | 1 | 2016 ControlEverything.com | PULL-UP | I2C 5V | ADS7828 | I2C IN | I2C OUT | MCP23008 | GND | +5V | SDA | SCL | SCL | SDA | +5V | +5V | GND | I2CCMR8x | REV.A | A1 | A0 | A1 | A1 | A0 | A2 | ADC / Address | Relay Address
